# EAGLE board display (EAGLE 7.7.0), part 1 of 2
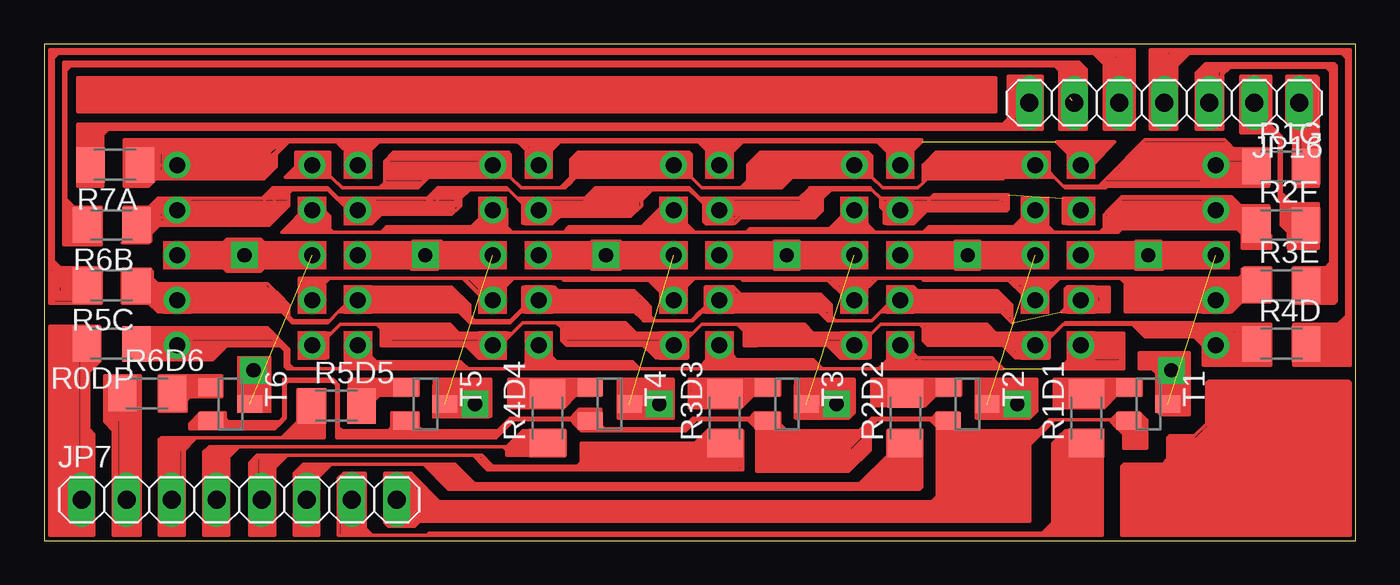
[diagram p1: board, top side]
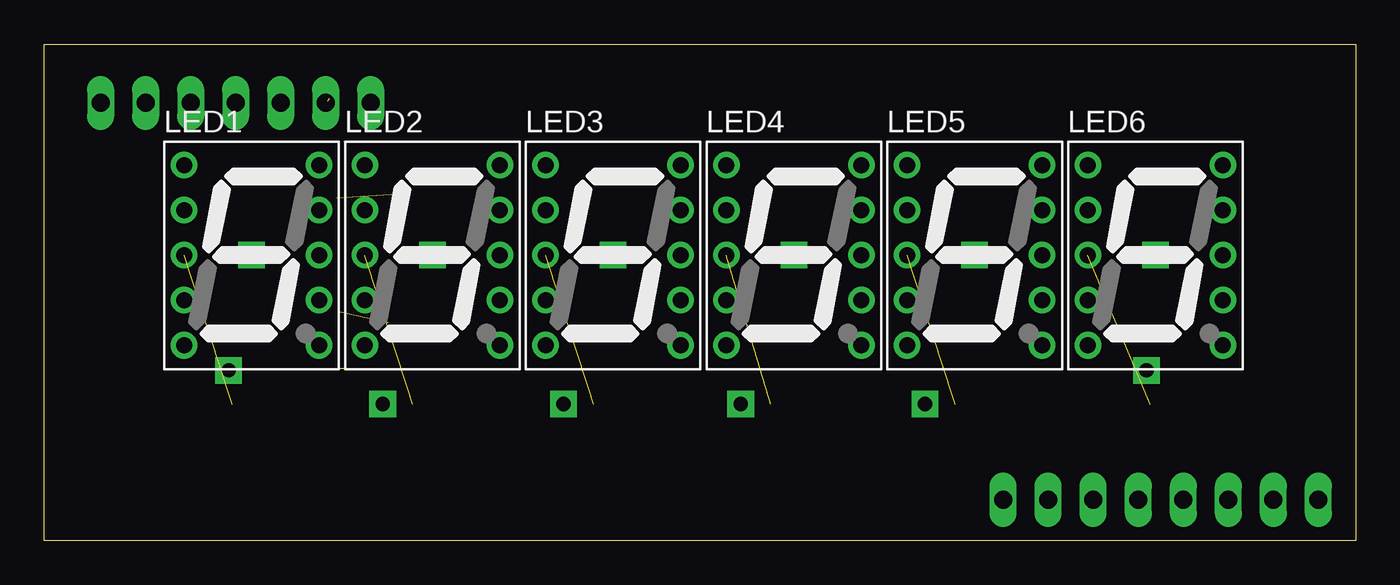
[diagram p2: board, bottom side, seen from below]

Size 74 x 28 mm. Coordinates in mm from the lower left corner, seen from the top.
Outline: 0,0 74,0 74,28 0,28 0,0
Copper layers (1*16): Top 0.035mm / dielectric 1.5mm / Bottom 0.035mm
Design rules "default": minimum track width 10mil, minimum drill 24mil, track to track 8mil, track to pad 8mil, pad to pad 8mil, via to via 8mil, smd to smd 8mil, copper to edge 40mil, drill to drill 8mil, minimum pad ring 10mil, minimum via ring 8mil, stop-mask expansion 4mil, vias tented up to drill 0mil, thermal gap 10mil

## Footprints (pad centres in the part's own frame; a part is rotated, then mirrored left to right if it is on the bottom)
1X08 = drill 1.016 long: 1 -8.89,0; 2 -6.35,0; 3 -3.81,0; 4 -1.27,0; 5 1.27,0; 6 3.81,0; 7 6.35,0; 8 8.89,0
1X07 = drill 1.016 long: 1 -7.62,0; 2 -5.08,0; 3 -2.54,0; 4 0,0; 5 2.54,0; 6 5.08,0; 7 7.62,0
SA39-11SRWA = drill 0.9 pad 1.5: 1 -3.81,5.08; 2 -3.81,2.54; 3 -3.81,0; 4 -3.81,-2.54; 5 -3.81,-5.08; 6 3.81,-5.08; 7 3.81,-2.54; 8 3.81,0; 9 3.81,2.54; 10 3.81,5.08
M1206 = smd 1.6 x 2: 1 -1.4,0; 2 1.4,0
SOT23-BEC = smd 1 x 1.4: B -0.95,-1.1; C 0,1.1; E 0.95,-1.1

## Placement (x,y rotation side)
JP7  [1X08]  11,2.3 0 top
JP16  [1X07]  63.2,24.7 180 top
LED1  SA39-11SRWA  [SA39-11SRWA]  62.3,16.1 0 bottom
LED2  SA39-11SRWA  [SA39-11SRWA]  52.1,16.1 0 bottom
LED3  SA39-11SRWA  [SA39-11SRWA]  41.9,16.1 0 bottom
LED4  SA39-11SRWA  [SA39-11SRWA]  31.7,16.1 0 bottom
LED5  SA39-11SRWA  [SA39-11SRWA]  21.5,16.1 0 bottom
LED6  SA39-11SRWA  [SA39-11SRWA]  11.3,16.1 0 bottom
R0DP  [M1206]  3.8,11.1 180 top
R1D1  4k7  [M1206]  58.8,6.9 90 top
R1G  [M1206]  69.8,21.1 0 top
R2D2  4k7  [M1206]  48.6,6.9 90 top
R2F  [M1206]  69.8,17.8 0 top
R3D3  4k7  [M1206]  38.4,6.9 90 top
R3E  [M1206]  69.8,14.4 0 top
R4D  [M1206]  69.8,11.1 0 top
R4D4  4k7  [M1206]  28.4,6.9 90 top
R5C  [M1206]  3.8,14.4 180 top
R5D5  4k7  [M1206]  16.5,7.6 0 top
R6B  [M1206]  3.8,17.8 180 top
R6D6  4k7  [M1206]  5.8,8.3 0 top
R7A  [M1206]  4,21.2 180 top
T1  [SOT23-BEC]  62.3,7.7 270 top
T2  [SOT23-BEC]  52.1,7.7 270 top
T3  [SOT23-BEC]  41.9,7.7 270 top
T4  [SOT23-BEC]  31.9,7.7 270 top
T5  [SOT23-BEC]  21.5,7.7 270 top
T6  [SOT23-BEC]  10.5,7.7 270 top

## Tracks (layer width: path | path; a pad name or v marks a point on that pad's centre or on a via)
N$1
  Top 0.2: T1.B 59.05,8.65 58.8,8.4 R1D1.2
N$2
  Top 0.2: T2.B 48.85,8.65 48.6,8.4 R2D2.2
N$3
  Top 0.2: T3.B 38.65,8.65 38.4,8.4 R3D3.2
N$4
  Top 0.2: T4.B 28.65,8.65 28.4,8.4 R4D4.2
N$5
  Top 0.2: T5.B 18.25,8.65 18,8.4 R5D5.2
N$6
  Top 0.2: 5.6,22.1 6.4,22.1 6.7,21.8 6.7,20.5 6.1,20.5 6,20.4 6,21.8 6.1,21.9 6.3,21.9 | 6.3,21.9 6.4,21.9 6.5,21.8 6.5,20.8 6.6,20.7 6.3,20.7 6.2,20.6 6.2,20.9 | 6.2,20.9 6.2,21.1 | 6.2,21.8 6.2,21.1 | 6.2,21.1 6.4,20.9 6.4,21.8 6.3,21.9 | 6.6,20.8 6.3,20.8 6.2,20.9
N$7
  Top 0.2: 30.4,8.9 26.4,8.9 26.3,9 26.3,8.8 30.2,8.8 30.3,8.7 30.3,8.6 30.2,8.5 26.5,8.5 26.4,8.6 27.8,8.6 27.9,8.7 26.3,8.7 26.2,8.6 | 26.2,8.6 26.2,9.1 31.4,9.1 31.3,9 31.4,8.9 31.4,8.2 30,8.2 29.3,7.5 26.3,7.5 26.2,7.6 26.2,7.7 | 26.2,8.6 26.2,7.7 | 26.2,7.7 26.3,7.6 27.3,7.6 27.4,7.7 26.4,7.7 26.3,7.8 27.4,7.8 27.4,7.9 27.5,8 26.3,8 26.3,8.2 27.5,8.2 27.5,8.3 26.3,8.3 26.3,8.4 26.4,8.5 30,8.5 30.1,8.4 29.4,8.4 29.3,8.3 29.3,8.2 | 29.3,7.9 29.2,7.8 29.5,7.8 30,8.3 29.8,8.3 | 29.5,8.3 29.4,8.3 29.3,8.2 | 29.3,8.2 29.3,8.1 | 29.3,8.1 29.3,7.9 | 29.3,7.9 29.4,7.9 29.8,8.3 | 29.8,8.3 29.7,8.3 | 29.7,8.3 29.5,8.3 | 29.5,8.3 29.3,8.1 | 29.3,8.1 29.5,8.1 29.7,8.3
N$9
  Top 0.2: 5.9,18.7 6,18.7 6.5,19.2 6.6,19.2 6.7,19.1 | 6.7,19.1 6.6,19.1 5.9,18.4 6,18.4 6.7,19.1 | 6.7,19.1 6.7,18.2 6.6,18.2 6,17.6 6,17.8 | 6,18 6,18.2 6.6,18.8 6.6,18.5 6.5,18.4 6.5,18.3 6,17.8 | 6,17.8 6,18 | 6,18 6.5,18.5
N$10
  Top 0.2: 12.3,22.3 13.3,22.3 13.3,22.2 | 13.3,22.2 12.6,21.5 12.6,22.2 13,22.2 | 13.3,22.2 13,22.2 | 13,22.2 12.7,21.9 | 12.7,21.9 12.7,22.1 | 12.7,21.9 12.7,21.4 | 12.7,21.4 12.6,21.3 12.6,20.8 12.5,20.7 12.5,21.5 12.7,21.5 12.9,21.7 12.9,21.1 12.7,20.9 12.7,21.4 | 12.7,21.4 12.8,21.5
N$11
  Top 0.2: R4D.1 68.4,11.02 LED1.5 66.11,11.95 65.86,12.2 61.8,12.2 | 39.5,11.27 39.75,11.02 LED3.5 46.4,11.7 46.6,11.6 | 36.1,11.27 36.15,11.02 LED4.5 29.45,11.02 29.2,11.27 29.2,12 28.9,12.3 | LED5.5 19.25,11.02 19,11.27 | 19,11.27 19,11.95 18.75,12.2 | LED6.5 15.52,11.02 15.8,11.3 | 18.75,12.2 16.7,12.2 16.2,11.7 | 16.2,11.7 16,11.5 | 16,11.5 15.8,11.3 | 15.8,11.3 15.8,11.7 16.2,11.7 | 16,11.5 16,10.3 15.8,10.3 15.7,10.4 | 18.75,12.2 22.9,12.2 23.4,11.7 26,11.7 | 19,11.27 19,11 23.8,11 24.5,10.3 26,10.3 26,11.3 27,12.3 28.9,12.3 | 25.6,11.5 25.8,11.5 26,11.7 | 26,11.7 26.2,11.7 | 26.3,11.7 26.2,11.7 | 26.2,11.7 26.1,11.6 | 28.9,12.3 32.8,12.3 33.4,11.7 | 33.5,11.6 33.4,11.7 | 33.4,11.7 36.6,11.7 | 39.5,11.3 39.5,11.27 | 35.9,11.6 36.3,11.6 | 36.3,11.6 36.4,11.6 | 39.5,11.3 39.6,11.1 45.2,11.1 45.3,11.2 39.7,11.2 39.6,11.3 44.1,11.3 45.1,10.3 45.1,10.5 44.7,10.9 45,10.9 45,10.3 44.9,10.3 44.2,11 | 39.5,11.3 39.5,11.8 | 39.5,11.8 39.5,11.9 39.1,12.2 | 29.2,12.2 32.7,12.2 33.4,11.5 34.8,11.5 34.8,11.2 33.6,11.2 | 33.6,11.2 29.5,11.2 29.4,11.3 29.4,11.5 | 29.4,11.6 29.4,11.9 29.3,12 32.6,12 32.7,12.1 32.7,12 32.8,11.9 | 32.8,11.9 33,11.7 | 29.4,11.5 33.2,11.5 33,11.7 | 29.4,11.5 29.4,11.6 | 29.4,11.6 29.5,11.7 33,11.7 | 32.8,11.9 29.5,11.9 29.5,11.4 34.8,11.4 34.9,11.3 | 33.6,11.2 34.5,10.3 36.3,10.3 36.3,10.8 | 36.3,10.8 36.1,11.1 36,11.4 36.1,11.5 36.4,11.6 | 36.4,11.6 36.2,11.4 | 36.2,11.4 36.2,11.2 | 36.2,11.2 36.3,11.1 36.3,11.3 36.2,11.5 36.2,11.4 | 36.2,11.2 36.1,11.2 | 36.1,11.2 35.5,11.2 34.7,10.4 34.6,10.4 34.1,10.9 34.7,10.9 34.8,10.8 34.8,10.7 | 34.8,10.7 34.7,10.6 34.5,10.6 34.3,10.8 34.7,10.8 34.8,10.7
  Top 0.2: 36.4,11.6 36.5,11.6 | 36.6,11.7 37.1,12.2 39.1,12.2 | 36.6,11.7 36.1,11.2 | 36.3,11.6 36.3,10.8 | 39.1,12.2 42.9,12.2 43.4,11.7 46.7,11.7 | 39.1,12.2 39.5,11.8 | 39.5,11.27 39.5,11 40.2,11 | 46.6,11.6 46.7,11.7 | 49.4,12.2 47.2,12.2 46.7,11.7 | 49.4,12.2 49.6,12 49.6,11.27 49.85,11.02 LED2.5 55.93,11 56.3,11 57,11.7 | 46.6,11.6 46.4,11.2 46.4,11.4 46.6,11.6 | 46.6,11.6 46.6,10.3 46.2,10.3 46.1,10.4 | 49.4,12.2 53.2,12.2 53.7,11.7 | 53.8,11.6 53.7,11.7 | 53.7,11.7 56.6,11.7 | 56.6,11.7 56.6,11.5 | 56.6,11.5 56.6,11.4 55.5,10.3 54.8,10.3 54.1,11 55,11 55.2,10.8 55.2,10.5 55.1,10.4 54.9,10.4 54.4,10.9 55,10.9 55.1,10.8 55.1,10.7 55,10.6 54.8,10.8 54.7,10.8 54.7,10.7 55.1,11.1 | 57,11.7 57.5,12.2 | 57.5,12.2 61.4,12.2 | 61.4,12.2 61.8,12.2 | 56.6,11.7 56.8,11.7 | 57,11.7 56.8,11.7 | 56.8,11.7 56.7,11.6 | 56.6,11.5 56.7,11.6 | 56.7,11.6 56.7,10.3 56.1,10.3 56,10.4 | 61.8,12.2 62,12 | 62.1,11.9 62.3,11.7 64.7,11.7 65.4,11 65.4,9.9 69.2,9.9 69.2,10.1 | 69.2,12.1 66,12.1 65.9,12.2 69.1,12.2 | 69.1,12.2 69.2,12.1 | 69.2,12.1 69.2,10.1 | 69.2,10.1 69.1,10 65.7,10 65.6,10.1 | 65.6,10.1 65.5,10.1 | 65.6,10.1 67.4,10.1 67.6,10.3 | 67.6,10.3 67.6,10.1 | 67.6,10.3 67.6,11.9 62.1,11.9 | 62.1,11.9 62,12 | 62,12 67.1,12 67.3,11.8 | 67.3,11.8 67.4,11.7 67.5,11.7 67.5,10.3 67.4,10.2 67,10.2 66.9,10.3 66.9,10.5 | 66.9,11.8 66.9,10.5 | 66.9,10.5 67.1,10.3 67.1,11.7 67,11.8 67,10.6 67.2,10.4 67.2,11.7 67.3,11.8 | 67.3,11.8 67.3,11.7 67.4,11.6 67.4,10.4 67.3,10.3 66.3,10.3 64.8,11.8 65,11.8 | 65.2,11.8 65.3,11.8 | 65.3,11.8 65.4,11.7 65.4,11.6 | 65.4,11.6 65.3,11.5 65,11.8 | 65,11.8 65.2,11.8 | 65.2,11.8 65.4,11.6 | 57.5,12.2 57.6,12.3 64.8,12.3 65.3,11.8
  Top 0.2: 69.1,12.2 69.2,12.2 69.2,12.1 | 61.4,12.2 62.1,11.5 65.7,11.5 65.8,11.4
N$12
  Top 0.2: 28.4,10.6 29,10
N$13
  Top 0.2: 37.8,19 37.4,19 37.2,19.2
N$14
  Top 0.2: 72.8,15.6 72.8,26.7 72.7,26.8 72.5,26.8 | 72.4,26.8 72.5,26.8 | 72.5,26.8 72.7,26.6
N$15
  Top 0.2: 38.7,10.7 38.7,10.6 39.2,10.1
N$16  (1 unrouted)
  Top 0.2: LED1.8 LED1.3
N$17  (1 unrouted)
  Top 0.2: 55.99,16.44 LED2.3 LED2.8
N$18
  Top 0.2: 13.7,12.7 13.7,13.3 13.6,13.3 | 13.6,13.3 13.6,13 | 13.6,12.8 13.6,13 | 13.6,13 6.5,13 6.1,13.4 6.3,13.4 | 6.3,13.4 13.5,13.4 13.6,13.3 | 13.6,13.3 6.4,13.3 6.3,13.4 | 6.3,13.4 6.3,13.3 6.4,13.2 13.4,13.2 13.5,13.1 13.5,13.3 12.8,14 | 12.7,14.1 12.5,14.3 6.4,14.3 6,14.7 6,14 | 6,14 6,13.8 6.1,13.7 13,13.7 | 13,13.7 13.2,13.5 | 13,13.7 12.8,13.9 6,13.9 5.9,14 6,14 | 6,14 6.1,14 | 6.1,14 12.8,14 | 12.8,14 12.7,14.1 | 12.7,14.1 6.3,14.1 6.2,14.2 6.2,14.3 6.1,14.4 6.1,14 | 6.1,14 6.3,14.2
N$19
  Top 0.2: 10.45,5.3 10.2,5.05 10.2,2.87 JP7.4 | 10.45,5.3 11,5.3 | 11,5.3 25.9,5.3 | 25.9,5.3 26.1,5.3 | 26.2,5.3 26.4,5.3 | 26.4,5.3 26.5,5.3 | 26.5,5.3 26.8,5.3 | 26.8,5.3 27.3,5.3 27.5,5.5 R4D4.1 | 9.4,5.3 9.3,5.3 9,5 9,0.8 | 9,0.8 10.4,0.8 | 10.4,0.8 10.4,4.7 11,5.3 | 10.45,5.3 9.4,5.3 | 9.4,5.3 9.1,5 9.2,5 | 9.2,5 9.3,5 | 9.3,5 9.5,5 | 9.7,5 10.5,5 | 10.5,5 10.7,5.2 9.4,5.2 9.2,5 | 10.5,5 10.3,4.8 10.3,1 10.2,0.9 10.1,0.9 10.1,4.9 9.9,4.9 9.9,0.9 9.7,0.9 9.7,5 | 9.7,5 9.5,5 | 9.5,5 9.5,0.9 9.4,0.9 9.4,4.9 9.3,5 | 9.3,5 9.3,1 9.2,0.9 9.2,5 | 9,0.8 9,0.3 10.4,0.3 10.4,0.5 | 10.4,0.8 10.4,0.5 | 10.4,0.5 10.3,0.4 9.2,0.4 9.1,0.5 9.1,0.6 10.3,0.6 | 26.1,5.3 27,6.2 29.4,6.2 29.4,4.8 26.1,4.8 26.1,5.1 25.9,5.3 | 26.1,5.3 26.2,5.3 | 26.2,5.3 27,6.1 27.3,6.1 27.3,4.9 26.4,4.9 26.2,5.1 | 26.2,5.1 26.2,5.2 | 26.2,5.1 26.2,4.9 27,4.9 27.2,5.1 27.2,5.9 27,5.9 26.4,5.3 | 26.4,5.3 26.4,5 27,5 27.1,5.1 27.1,5.8 27,5.8 26.5,5.3 | 26.5,5.3 26.5,5.1 26.9,5.1 26.9,5.5 27,5.6 27,5.5 26.8,5.3 | 26.8,5.3 26.8,5.4
N$20
  Top 0.2: 13.7,6 15.7,6 15.7,6.1 15.8,6.2 | 15.2,7.9 15.2,8.5 14.3,8.5 14.3,6.7 13.4,5.8 | 13.4,5.8 8.25,5.8 8,5.55 8,5.3 7.85,5.3 7.49,4.94 JP7.3 | 13.4,5.8 15.1,5.8 | 15.1,5.8 R5D5.1 | 15.1,5.8 15.8,5.8 15.8,6.2 | 15.8,6.2 15.8,8.5 | 15.8,6.2 14,6.2 | 14,6.2 13.7,5.9 | 14,6.2 14.4,6.6 15.7,6.6 15.7,6.3 14.2,6.3 14.4,6.5 15.5,6.5 15.6,6.4
N$21
  Top 0.2: R6D6.1 4.4,3.55 4.65,3.3 4.7,3.3 4.95,3.05 JP7.2
N$22
  Top 0.2: 14.5,21.1 14.4,21.1 13.9,20.6 14.4,20.6 14.2,20.8
N$23
  Top 0.2: 17,22.1 18.3,22.1 18.6,22.4 17,22.4 17,22.3 17.1,22.2 18.2,22.2 18.3,22.3
N$24
  Top 0.2: 5.9,17.5 6,17.5 6.5,18 6.7,18
N$25  (1 unrouted)
  Top 0.2: LED6.8 7.73,16.46 7.73,16.35 7.98,16.1 LED6.3
N$26
  Top 0.2: T6.B 8.05,8.65 7.8,8.4 R6D6.2
N$27  (1 unrouted)
  Top 0.2: 45.83,16.46 LED3.3 LED3.8
N$28
  Top 0.2: 14.8,1.3 14.8,0.8 | 14.8,0.8 14.7,0.8 | 14.7,0.8 14.1,0.8 | 14.1,0.8 14.1,3.8 14.6,4.3 15.1,4.3 | JP7.6 15.1,2.71 | 15.1,3.8 15.1,3.9 | 15.1,3.9 15.1,4.1 | 15.1,4.1 15.1,4.3 | 15.1,4.3 15.3,4.3 | 15.3,4.3 16,4.3 | 16.2,4.3 21.4,4.3 | 21.4,4.3 23.1,4.3 | 23.1,4.3 23.15,4.3 23.4,3.85 23.4,3.2 | 23.4,3.2 23.4,2.9 | 23.4,2.9 24.5,2.9 | 24.5,2.9 48.35,2.9 48.6,3.15 R2D2.1 | 15.3,4.3 15.1,4.1 | 15.1,2.71 15.1,1.2 | 15.1,1.2 14.7,0.8 | 14.8,0.8 15.5,0.8 | 15.5,0.8 15.5,3.6 16.2,4.3 | 16.2,4.3 16,4.3 | 16,4.3 15.8,4.1 14.6,4.1 14.6,4 14.3,3.7 14.3,3.8 14.4,3.9 14.4,4 14.5,4.1 15.6,4.1 15.7,4 14.8,4 14.7,3.9 14.7,3.7 | 14.7,3.7 14.7,1 14.6,0.9 14.3,0.9 14.3,3.6 14.6,3.9 15.1,3.9 | 15.1,3.9 15.5,3.9 | 15.6,3.9 15.5,3.9 | 15.5,3.9 15.4,3.8 15.4,1 15.3,0.9 15.3,1 | 15.3,1 15.3,3.5 15.6,3.8 15.2,3.8 | 15.2,3.8 15.1,3.8 | 15.1,3.8 15.1,2.71 | 15.1,1.2 15.3,1 | 15.3,1 15.1,1 15,0.9 15,3.8 15.1,3.9 | 15.1,3.9 15.2,3.8 | 15.2,3.8 15.2,1.3 15.1,1.2 | 15.1,1.2 14.9,1.2 14.9,3.8 14.8,3.8 14.7,3.7 | 14.7,3.7 14.5,3.7 14.5,1 | 14.2,1.2 14.2,0.9 14.1,0.8 | 14.1,0.8 14.1,0.3 15.5,0.3 15.5,0.5 | 15.5,0.8 15.5,0.5 | 15.5,0.5 14.2,0.5 14.2,0.6 15.3,0.6 15.4,0.7 | 21.4,4.3 22.8,2.9 23.4,2.9 | 23.1,4.3 24.5,2.9 | 24.5,2.9 24.5,3 23.2,4.3 21.8,4.3 21.7,4.2 22.9,3 24.2,3 | 24.2,3 24.2,3.1 24.1,3.2 | 24.1,3.2 23.4,3.2 | 23.4,3.2 23,3.2 22.9,3.1 22.9,3.2 21.9,4.2 23,4.2 23.9,3.3 23.7,3.3 | 23.2,3.3 23,3.3 22.2,4.1 22.9,4.1 23.7,3.3 | 23.7,3.3 23.5,3.3 | 23.3,3.3 23.2,3.3 | 23.2,3.3 22.5,4 22.8,4 23.5,3.3 | 23.5,3.3 23.3,3.3 | 23.3,3.3 22.7,3.9 | 24.2,3 46,3 47.7,4.7 | 24.1,3.2 46,3.2 47.7,4.9
N$29
  Top 0.2: 67.1,26.8 67,26.8 66.3,26.1
N$31
  Top 0.2: R2F.2 69.9,17.8 | 69.8,18 69.8,19.6 | 69.8,19.6 69.8,22.75 | 69.8,22.75 69.45,23.1 69.3,23.1 | 68.3,24.68 68.3,23.1 69.3,23.1 | 68.3,24.68 JP16.2 | 69.8,17.8 69.9,17.8 | 69.9,17.8 70.2,17.5 70.2,17.4 | 70.2,17.4 70.2,17.1 | 70.2,17.1 70.2,17 | 70.2,17 70.4,16.8 70.5,16.8 | 71.8,16.8 71.9,16.8 | 71.9,16.8 71.9,16.9 | 71.9,16.9 71.9,19 70.4,19 70.3,19.1 | 70.2,19.2 69.9,19.5 69.9,18.1 70,18 | 70,18 70.4,17.6 70.4,17.1 70.3,17 70.3,17.2 | 70.3,17.2 70.3,17.5 69.8,18 | 69.8,18 69.8,17.8 | 69.8,17.8 70.2,17.4 | 70,19.2 70,18.7 | 70,18.7 70,18 | 70,18 70.2,18 | 70.2,18 70.3,17.9 70.3,18.9 | 70.3,18.9 70.3,19.1 | 70.3,19.1 70.2,19.2 | 70.2,19.2 70.2,18.8 | 70.2,18 70.2,18.8 | 70.2,18.8 70.3,18.9 | 70.3,18.9 71.7,18.9 71.8,18.8 | 70.1,19.2 70.1,19.3 69.8,19.6 | 69.3,23.1 69.4,23 | 69.4,23 69.7,22.7 69.7,19.2 70,18.7 | 69.4,23 67.6,23 | 67.6,23 67.6,23.2 | 67.6,25.9 67.6,26.2 69.2,26.2 69.2,23.4 69.8,22.8 69.8,22.75 | 67.6,23 67.5,23 67.5,26.2 69,26.2 69.1,26.1 69.1,23.3 69.2,23.2 67.6,23.2 | 67.6,23.2 67.6,25.9 | 67.6,25.9 67.8,26.1 69,26.1 69,23.3 68,23.3 67.8,23.5 67.7,23.4 68.8,23.4 68.9,23.5 68.9,26 67.9,26 67.8,25.9 67.8,23.6 67.7,23.5 68.7,23.5 68.7,25.9 68,25.9 | 68,25.9 67.9,25.9 67.9,23.7 68.6,23.7 68.6,25.8 68.1,25.8 68,25.9 | 68,25.9 68,23.9 68.1,23.9 | 68.4,23.9 68.5,23.8 68.5,25.6 68.4,25.7 68.3,25.7 | 68.3,25.7 68.1,25.7 68.1,23.9 | 68.1,23.9 68.4,23.9 | 68.4,23.9 68.4,25.6 68.3,25.7 | 68.3,25.7 68.3,24.68 | 70.3,17.2 70.2,17.1 | 70.2,17 70.2,16.5 71.9,16.5 71.9,16.7 | 71.9,16.7 71.8,16.8 | 71.8,16.8 70.5,16.8 | 70.5,16.8 70.3,16.6 71.8,16.6 71.8,16.8 | 71.8,16.8 71.9,16.9 | 71.9,16.8 71.9,16.7
N$32
  Top 0.2: R1G.2 71.2,23.55 70.95,23.8 70.95,24.57 JP16.1
N$33
  Top 0.2: 4,1.7 4.6,1.7 4.6,1 | 4.6,0.8 3.9,0.8 | 3.9,0.8 3.9,6.2 | 3.9,6.5 3.9,6.6 | 3.9,6.6 3.9,6.8 | 3.9,6.8 3.9,7.1 3.4,7.1 | 3.4,7.1 3.4,7.4 | 3.4,7.4 3.4,9.3 3.6,9.3 | 5.2,9.3 5.2,9.2 5.4,9.2 | 5.4,9 5.4,0.8 | 5.4,0.8 4.6,0.8 | 4.6,0.8 4.6,1 | 4.6,1 4.8,1 | 4.9,1 5,1 | 5.1,1 5.2,1 | 5.2,1 5.3,1 5.3,9 5.4,9 | 5.4,9 5.4,9.2 | 5.4,9.2 5.4,9.3 5.2,9.3 | 5.2,9.3 3.6,9.3 | 3.6,9.3 3.6,7.3 | 4.1,7.3 5.2,7.3 5.2,7.1 | 5.2,7.1 3.6,7.1 3.6,7.3 | 3.6,7.3 3.7,7.3 | 3.7,7.3 4.1,7.3 | 4.1,7 4.1,0.9 4.3,0.9 4.3,6.9 4.2,6.9 4.2,7 4.1,7 | 4.1,7 4.1,7.3 | 3.6,7.3 3.5,7.3 | 3.5,7.2 3.5,7.3 | 3.5,7.3 3.4,7.4 | 3.4,7.1 3.4,6.8 | 3.4,6.8 3.4,6.7 3.9,6.2 | 3.9,6.2 3.9,6.5 | 3.9,6.5 3.6,6.8 3.6,6.9 3.5,7 3.7,7 3.9,6.8 | 3.9,6.8 4.7,6.8 | 4.7,6.8 4.9,6.8 | 4.9,6.8 5.1,6.8 5.2,6.9 5.1,7 4.6,7 4.5,6.9 4.5,1.1 4.4,1 4.6,1 | 5.2,1 5.2,7.1 | 5.2,7.1 5.1,7.2 5.1,1 | 5.1,1 5,1 | 5,1 5,6.7 4.9,6.8 | 4.9,6.8 4.9,1 | 4.9,1 4.8,1 | 4.8,1 4.7,1.1 4.7,6.8 | 3.7,7.3 3.7,6.8 3.9,6.6 | 3.9,6.6 3.6,6.6 3.4,6.8 | 3.4,6.8 3.5,6.8 4,6.3 | 3.9,0.8 3.9,0.6 | 3.9,0.6 3.9,0.4 | 3.9,0.4 5.4,0.4 | 5.4,0.4 5.4,0.5 5.4,0.6 | 5.4,0.6 5.4,0.8 | 5.4,0.6 3.9,0.6 | 3.9,0.4 3.9,0.3 5.4,0.3 5.4,0.4
N$34
  Top 0.2: R0DP.2 JP7.1
N$35  (1 unrouted)
  Top 0.2: LED4.8 LED4.3
N$36
  Top 0.2: 7,8.9 6.5,8.9 6.5,9.3 10,9.3 10,8.1 8.2,8.1 8,7.9 8,7.3 6.5,7.3 6.5,8.8 6.7,9
N$37
  Top 0.2: 7.7,9.1 9.9,9.1 9.8,9 7.8,9 | 7.7,9 7.8,9 | 7.8,9 8,8.8 8.8,8.8 8.8,8.6 8.2,8.6 8,8.4 8,8.3 | 8,8.3 7.7,8 7.9,8 8.4,8.5 8.9,8.5 8.7,8.3 8,8.3 | 7.8,8.3 8,8.3 | 8,8.3 8.2,8.5
N$38
  Top 0.2: 12.7,14.2 13.3,13.6
N$39
  Top 0.2: 45.2,11.5 39.5,11.5 39.5,11.9 39.4,12 43,12 43,11.9 43.3,11.6 39.7,11.6 39.6,11.7 43.1,11.7 42.9,11.9 39.7,11.9 39.6,11.8 39.6,11.4 39.5,11.3
N$40
  Top 0.2: 6.8,2.6 6.5,2.6 | 6.5,2.6 6.5,5.7 6.6,5.8 8.2,5.8 | 6.5,2.6 6.5,0.8 | 6.5,0.8 7.9,0.8 | 7.9,0.8 7.9,5.1 8.5,5.7 6.6,5.7 6.6,0.9 7.8,0.9 7.8,5.1 8.3,5.6 6.8,5.6 6.7,5.5 6.7,1 7,1 | 7.2,1 7.5,1 7.6,1.1 7.6,5.2 7.9,5.5 6.9,5.5 6.9,1.2 6.8,1.1 7.3,1.1 | 7.3,1.1 7.5,1.1 7.5,5.3 7.6,5.4 7.3,5.4 | 7.3,5.4 7.1,5.4 7.1,1.1 7,1 | 7,1 7.2,1 | 7.2,1 7.3,1.1 | 7.3,1.1 7.3,5.4 | 6.5,0.8 6.5,0.3 7.9,0.3 7.9,0.7 | 7.9,0.8 7.9,0.7 | 7.9,0.7 7.8,0.6 6.6,0.6 6.6,0.5 7.6,0.5 7.7,0.4 7.8,0.5
N$41
  Top 0.2: 24.5,4.7 24.9,4.3 25,4.3
N$42
  Top 0.2: 24.7,4.4 24.7,4.3 25,4 38.8,4 39.4,4.6 | 39.4,4.6 39.4,4.7 | 39.4,4.7 39.4,6.2 37.4,6.2 36.7,5.5 | 13.05,4.8 12.8,4.55 12.8,3.9 | 13.05,4.8 13.2,4.8 | 13.2,4.8 13.5,4.8 | 13.7,4.8 24.2,4.8 | 24.2,4.8 24.7,4.8 | 24.7,4.8 24.8,4.6 25.2,4.3 | 25.2,4.3 25.3,4.2 | 25.3,4.2 30.3,4.2 | 30.3,4.2 30.6,4.2 | 30.6,4.2 30.8,4.2 30.8,5.3 31,5.5 36.7,5.5 | 36.9,5.5 R3D3.1 | JP7.5 12.8,2.93 12.8,3.9 | 12.2,4.8 12,4.8 11.6,4.4 11.6,0.8 | 11.6,0.8 11.9,0.8 | 13,0.8 13,4.3 | 13,4.4 13,4.6 13.2,4.8 | 13.05,4.8 12.2,4.8 | 12.2,4.8 12,4.6 | 12,4.6 11.7,4.3 11.7,0.9 12,0.9 | 12.3,0.9 12.9,0.9 12.9,4.6 12.8,4.7 12.6,4.7 | 12.4,4.7 12.2,4.7 12.2,0.9 | 12.2,0.9 12,0.9 | 12,0.9 12,4.6 | 12,4.6 11.9,4.6 11.8,4.5 11.8,1 12.1,1 12.2,0.9 | 12.2,0.9 12.3,0.9 | 12.3,0.9 12.4,1 12.4,4.7 | 12.4,4.7 12.6,4.7 | 12.6,4.7 12.6,1.1 12.5,1 12.7,1 12.7,4.1 | 12.8,3.9 13.7,4.8 | 13.7,4.8 13.5,4.8 | 13.5,4.8 13,4.3 | 13,4.3 13,4.4 | 13,4.4 13.3,4.7 | 11.6,0.8 11.6,0.3 13,0.3 13,0.8 | 13,0.8 11.9,0.8 | 11.9,0.8 11.7,0.6 12.9,0.6 12.9,0.5 11.8,0.5 11.7,0.4 | 24.2,4.8 24.8,4.2 25.3,4.2 | 24.7,4.8 25.2,4.3 | 36.7,5.5 36.9,5.5 | 36.9,5.5 37.4,6 37.4,5.9 37.1,5.6 37.4,5.6 37.4,5.7 | 39.3,5.1 39.3,4.8 39.4,4.7 | 39.4,4.6 39.4,4 38.7,4 38.6,4.1 39.1,4.1 39.3,4.3 39.3,4.2 | 30.3,4.2 30.3,5.5 31.2,5.5 31.3,5.4 30.6,5.4 30.5,5.3 30.5,5.1 30.5,4.6 | 30.5,4.6 30.5,4.3 30.6,4.2 | 30.6,4.2 30.6,5.1 30.7,5.2 30.5,5.2 30.4,5.3 | 31,5.3 31,4.7 | 31,4.7 31,4.3 30.8,4.1 31.1,4.1 | 31,4.7 30.4,4.1 30,4.1 30.5,4.6
N$43
  Top 0.2: 15.5,14.5 15.7,14.7
N$44  (1 unrouted)
  Top 0.2: LED5.8 LED5.3
N$45
  Top 0.2: 43.9,11.4 44.9,11.4 45,11.3
N$46
  Top 0.2: 18.4,14.1 23,14.1 23.4,13.7 | 23.5,13.6 23.9,13.2 18.1,13.2 17.8,13.5 23.5,13.5 23.7,13.3 18.5,13.3 18.5,13.7 23.4,13.7 | 23.4,13.7 23.5,13.6 | 23.5,13.6 23.3,13.6 23,13.9 18.4,13.9 18.4,13.1 23.8,13.1 23.9,13 17.9,13 17.8,12.9 23.6,12.9 24.1,12.4 24.1,12.6 23.8,12.9
N$47
  Top 0.2: 2.5,4.2 2.5,1 2.6,0.9 2.3,0.9 | 1.9,0.9 2.3,0.9 | 2.3,0.9 2.4,0.8 2.8,0.8 | 2.8,0.8 2.8,4.3 | 2.8,4.3 2.8,4.4 | 2.8,4.4 2.6,4.4 | 2.6,4.4 1.9,4.4 | 1.7,4.4 1.3,4.4 | 1.3,4.4 1.3,4.2 | 1.3,4.2 1.3,0.8 | 1.3,0.8 2.6,0.8 2.7,0.9 2.7,4.3 2.3,4.3 | 2.1,4.3 1.8,4.3 | 1.8,4.3 1.5,4.3 1.5,4.2 | 1.5,4.2 1.5,0.9 2,0.9 2.1,1 2,1.1 2,4 | 2.3,0.9 2.3,4.2 | 2.3,4.2 2.3,4.3 | 2.3,4.3 2.1,4.3 | 2.1,4.3 2,4.2 2,4 | 1.8,4.3 1.8,1.1 | 2.6,3.7 2.6,4.1 2.8,4.3 | 2.8,4.4 2.8,6 2.5,6.3 2.5,9.5 3.1,10.1 3.1,12.1 1.4,12.1 | 1.4,12.1 1.4,4.3 1.5,4.2 | 1.5,4.2 1.3,4.2 | 1.3,4.4 1.3,12.1 1.5,12.1 1.6,12 1.6,4.5 1.7,4.4 | 1.7,4.4 1.9,4.4 | 1.9,4.4 1.9,10.2 2,10.3 1.8,10.3 1.8,5.1 | 1.8,5.1 1.7,5 1.7,9.9 2.1,10.3 2.1,4.1 2,4 | 2,4 2.1,4 2.3,4.2 | 2.3,4.3 2.3,6.2 2.4,6.2 2.5,6.1 2.5,4.1 2.4,4 2.4,5.6 2.7,5.9 2.7,4.8 2.6,4.7 | 2.6,4.7 2.6,4.4 | 2.6,4.7 2.6,6 2.3,6.3 2.3,10 2.4,10.1 2.3,10.1 2.2,10 2.2,9.9 2.4,9.7 2.4,9.6 3,10.2 2.6,10.2 2.5,10.1 2.5,9.8 2.7,10 2.7,10.1 | 1.8,5.1 1.8,2.7 1.9,2.6 | 1.4,1 1.4,0.9 1.3,0.8 | 1.3,0.8 1.3,0.3 | 1.3,0.3 2.8,0.3 2.8,0.6 | 2.8,0.8 2.8,0.6 | 2.8,0.6 1.4,0.6 1.4,0.5 2.7,0.5 | 1.4,12.1 0.3,12.1 0.3,0.3 1.3,0.3
N$48
  Top 0.2: 2.1,3 2.1,1.2 2.2,1.1
N$49
  Top 0.2: 1.6,4.2 1.6,1.1 1.7,1
N$50
  Top 0.2: 20.8,3.2 20.9,3.2 22.1,2 22.1,1.7 21,1.7 21,2.8 21.1,2.9 21.1,2.8 22,1.9 21.2,1.9 21.1,1.8 21.1,2.5 21.2,2.6 21.2,2.1 21.3,2 21.6,2 | 21.7,2 21.6,2 | 21.6,2 21.3,2.3 21.4,2.4 21.4,2.3 | 21.4,2.3 21.6,2.1 | 21.4,2.3 21.3,2.4 21.3,2.1
N$51
  Top 0.2: 50.4,2.1 50.4,2.2 50.8,2.6 50.8,2.5 50.4,2.1
N$52
  Top 0.2: 53.8,1.5 54.2,1.5 54.3,1.6 54.1,1.6 53.9,1.4 54.1,1.4 55.5,2.8 55.5,2.9 | 55.5,2.9 55.5,6.1 54.6,6.1 54.5,6 54.5,2.1 | 54.5,1.9 54.5,2.1 | 54.5,2.1 55.4,3 55.4,3.2 | 55.4,5.9 55.4,6 | 55.4,6 54.7,6 54.7,2.4 54.6,2.3 54.6,2.4 55.4,3.2 | 55.4,3.2 55.4,5.9 | 55.4,5.9 54.9,5.9 54.8,5.8 54.8,2.9 | 54.8,2.7 54.8,2.9 | 54.8,2.9 55.3,3.4 55.3,5.4 | 55.3,5.4 55.3,5.8 55,5.8 54.9,5.7 54.9,3.3 55,3.2 55,5.6 55.1,5.7 55.1,3.4 | 36.4,6.6 36.4,6.7 36.6,6.9 39.8,6.9 40.1,7.2 41.5,7.2 41.5,6.6 41.9,6.2 | 31.3,7.2 30.1,7.2 30.1,7.1 30,7 | 30.7,6.8 30,6.8 | 30,6.8 30,7 | 30,7 30,7.2 | 30,7.2 30.2,7.4 31.4,7.4 31.4,6.5 31.7,6.2 | 19.8,3.5 19.8,3.8 19.2,3.8 19.2,1 19.4,0.8 20.6,0.8 | 20.6,0.8 20.6,3.8 | 20.6,3.8 19.5,3.8 19.4,3.7 19.4,1 19.5,0.9 19.7,0.9 | 19.9,0.9 20,0.9 | 20.2,0.9 20.3,0.9 20.4,1 | 20.4,1 20.4,3.6 20.5,3.7 20.2,3.7 | 20.2,3.7 19.7,3.7 | 19.7,3.7 19.6,3.7 19.5,3.6 19.5,1.1 19.6,1 20.4,1 | 20.4,1 20.5,0.9 20.5,3.4 20.2,3.7 | 20.2,3.7 20.2,0.9 | 20.2,0.9 20,0.9 | 20,0.9 20,3.6 19.9,3.6 19.8,3.5 | 19.8,3.5 19.8,1 19.9,0.9 | 19.9,0.9 19.7,0.9 | 19.7,0.9 19.7,3.7 | 20.6,3.8 20.7,3.8 20.9,3.6 | 20.9,3.4 20.9,1.1 | 20.9,1.1 20.9,0.8 | 20.9,0.8 20.6,0.8 | 20.6,0.8 20.7,0.9 20.7,3.6 | 20.9,0.8 21.3,1.2 54.1,1.2 55.6,2.7 | 9.1,7 8.9,7 8.8,7.1 | 8.8,7.1 8.8,7.2 | 8.8,7.2 10.1,7.2 | 10.1,7.2 10.1,7 | 10.1,7 10.1,6.4 10.2,6.3 | 10.1,7.2 10.2,7.2 10.2,6.4 | 10.2,6.4 10.2,6.3 | 10.2,6.3 8.2,6.3 8.2,6.6 8.8,7.2 | 8.8,7.1 8.8,7 8.3,6.5 8.8,6.5 8.7,6.6 8.6,6.6 | 8.5,6.6 8.6,6.6 | 8.6,6.6 8.7,6.7 | 9.9,6.6 10.5,6.6 | 10.5,6.6 13.3,6.6 | 13.3,6.6 13.6,6.9 13.6,8.9 13.7,9 13.5,9 | 19.6,6.9 19.75,6.75 T5.E 20.4,6.45 20.57,6.28 | 20.57,6.28 20.65,6.2 | 20.65,6.2 21.2,6.2
  Top 0.2: 21.2,6.2 25.85,6.2 26.1,6.45 26.1,6.65 26.35,6.9 | 26.35,6.9 26.6,6.9 | 26.6,6.9 29.7,6.9 | 29.7,6.9 30,6.9 30.15,6.75 T4.E 30.8,6.45 31.05,6.2 31.7,6.2 | 31.7,6.2 36.05,6.2 36.3,6.45 36.3,6.55 36.55,6.8 36.8,6.8 | 41.9,6.2 41.05,6.2 40.8,6.45 T3.E 40.05,6.75 40,6.8 | 41.9,6.2 46,6.2 | 46,6.2 46.15,6.2 46.4,6.45 46.4,6.55 46.65,6.8 | 51.6,6.2 51.25,6.2 51,6.45 T2.E 50.15,6.75 50.1,6.8 50,6.8 | 51.6,6.2 52.9,6.2 | 55.6,6.2 56.3,6.2 56.5,6.4 56.5,6.6 | 36.8,6.8 39.7,6.8 | 39.7,6.8 39.9,6.8 | 46.65,6.8 46.8,6.8 | 47,6.8 50,6.8 | 56.5,6.6 56.7,6.8 57,6.8 | 60.2,6.8 60.3,6.8 60.35,6.75 T1.E | 13.5,8.75 13.5,6.95 13.25,6.7 10.2,6.7 10.15,6.75 T6.E | 13.5,8.75 13.75,9 16.25,9 16.5,8.75 16.5,6.45 | 16.5,6.45 16.75,6.2 16.8,6.2 | 16.8,6.2 19.4,6.2 | 19.4,6.2 19.5,6.2 | 19.5,6.2 19.7,6.2 | 19.7,6.2 20.4,6.2 | 20.4,6.2 20.48,6.28 20.57,6.28 | 52.65,2.2 52.9,2.45 | 52.9,2.45 52.9,6.2 | 13.5,9 13.5,8.75 | 10.2,6.3 13,6.3 13.3,6.6 | 10.2,6.4 12.9,6.4 13,6.5 | 10.5,6.6 10.1,7 | JP7.8 20.6,2.3 20.6,1.5 52.9,1.5 52.9,2.45 | 55.6,2.7 55.6,5.6 | 55.6,5.6 55.6,6.2 | 55.6,6.2 52.9,6.2 | 51.6,6.2 51.6,7.2 50.4,7.2 50.1,6.9 50.1,6.7 | 50.1,6.7 50.3,6.5 | 50.3,6.9 50.3,6.5 | 50.3,6.5 50.4,6.4 | 50.4,6.4 50.5,6.3 50.5,2.4 50.3,2.2 22.3,2.2 20.9,3.6 | 20.9,3.6 20.9,3.4 | 20.9,3.4 22.2,2.1 22.2,1.4 21,1.4 21,1.1 21.2,1.3 22.2,1.3 22.3,1.4 | 20.65,6.2 20.4,6.2 | 19.7,6.2 19.7,7.2 | 19.7,7.2 19.6,7.2 19.6,6.3 19.5,6.2 | 19.7,7.2 21.1,7.2 21.1,6.3 21.2,6.2 | 16.5,6.45 16.5,5.8 25.5,5.8 26.1,6.4 | 19.9,6.5 19.7,6.5 19.4,6.2 | 25.7,6.1 25.8,6.1 26.6,6.9 | 16.6,6.2 16.6,6.1 | 16.6,6.1 16.6,6 25.5,6 25.6,6.1 25.5,6.1 | 25.5,6.1 21.4,6.1 | 21.4,6.1 16.6,6.1 | 20.9,6.6 21.4,6.1
  Top 0.2: 26.35,6.9 26.3,6.9 25.5,6.1 | 30,6.8 30,6.7 | 30,6.5 30.3,6.2 36.2,6.2 36.8,6.8 | 39.7,6.8 40.2,6.3 | 40.2,6.3 40.5,6 40.7,6 | 40.7,6 40.9,6.2 | 40.9,6.2 40.5,6.2 | 40.5,6.2 39.9,6.8 | 39.9,6.8 40,6.8 | 40,6.8 40.2,7 | 40.7,6 46.2,6 46.6,6.4 | 47,6.8 46.9,6.8 | 46.9,6.8 46.8,6.8 | 46.8,6.8 46.6,6.6 | 46.6,6.6 46.3,6.3 46.4,6.3 46.9,6.8 | 46.65,6.8 46.6,6.8 | 46.6,6.8 46,6.2 | 40.9,6.2 41.1,6.2 41.2,6.1 | 46.6,6.6 46.6,6.8 | 46.6,6.8 46.7,6.9 50.7,6.9 | 50,6.8 50.1,6.7 | 50.4,6.4 50.4,2.5 50,2.1 | 55.4,6 55.9,6 | 55.9,6 56.2,6 | 56.2,6 56.4,6.2 | 56.4,6.2 56.9,6.7 | 56.9,6.7 57,6.8 | 56.5,6.6 55.9,6 | 55.9,6 55.3,5.4 | 55.3,5.4 55.6,5.4 56.2,6 | 56.4,6.2 56.2,6.2 55.6,5.6 | 55.5,2.9 55.4,2.9 54.6,2.1 54.6,2.5 55,2.9 | 40.4,6.8 40.4,6.5 40.2,6.3 | 40.2,6.3 40.2,3.9 45.4,3.9 46.6,5.1 46.6,6.4 | 46.6,6.4 47,6.8 | 40.5,6.2 40.3,6 | 20.8,1.2 20.9,1.1 | 20.9,1.1 55.6,1.1 55.6,1.7 | 55.6,2.4 55.6,2.6 | 55.6,2.7 55.6,2.6 | 55.6,2.6 54.2,1.2 55.4,1.2 55.5,1.3 55.5,2.2 55.3,2.2 54.4,1.3 54.5,1.3 55.6,2.4 | 55.6,2.4 55.6,1.7 | 55.6,1.7 55.3,1.4 54.8,1.4 | 54.8,1.4 54.7,1.3 | 54.8,1.4 55.4,2 55.4,1.6 55.3,1.5 55.3,1.6 55.2,1.7 55.3,1.7 55.1,1.5 55.3,1.3 | 56.9,6.7 56.8,6.7 56.6,6.5 | 57,6.8 60.2,6.8 | 60.3,6.9 60.6,7.2 61.8,7.2 62.1,6.9 | 62.1,6.9 60.3,6.9 | 60.3,6.9 60.2,6.8 | 60.2,6.8 60.2,6.7 60.5,6.4 | 60.6,6.3 60.6,6.5 60.5,6.6 60.5,6.4 | 60.5,6.4 60.6,6.3 | 60.6,6.3 60.9,6 60.9,5.2 62.2,5.2 62.2,6.8 62.1,6.9 | 62.1,6.9 62,6.8 62,5.3 61.1,5.3 61,5.4 61,6.1 60.9,6.2 61.8,6.2 61.9,6.3 61.9,5.5 61.8,5.4 61.3,5.4 61.2,5.5 | 61.2,5.5 61.2,5.7 | 61.2,5.9 61.2,6.1 61.4,6.1 | 61.4,6.1 61.6,6.1 | 61.6,6.1 61.7,6 61.7,5.8 | 61.7,5.8 61.4,5.5 | 61.4,5.5 61.3,5.5 61.2,5.4 61.2,5.5
  Top 0.2: 61.2,5.8 61.2,5.9 | 61.2,5.9 61.4,6.1 | 61.6,6.1 61.7,6.1 61.8,6 61.8,5.7 | 61.8,5.7 61.8,5.5 61.4,5.5 | 61.4,5.5 61.2,5.7 | 61.2,5.7 61.2,5.8 | 61.2,5.8 61.4,6 61.5,6 61.7,5.8 | 61.3,5.8 61.7,5.8 | 61.7,5.8 61.8,5.7 | 61.8,5.7 61.7,5.6 61.4,5.6 61.3,5.7 | 26.4,6.8 29.7,6.8 30,6.5 | 30,6.5 30,6.7 | 30,6.7 29.9,6.8 29.8,6.8 29.7,6.9 | 29.7,6.9 30,7.2 | 13.5,9 13.5,9.1 16.3,9.1 16.6,8.8 16.6,6.4 16.8,6.2
N$53
  Top 0.2: 51.1,5.9 50.7,6.3 51,6.3 51.1,6.2
N$54
  Top 0.2: 50.7,5.9 50.7,6.1 50.6,6.2
N$55
  Top 0.2: 18.1,8.2 18.3,8.2 18.4,8.3 18.4,8.2 21.1,8.2 21.1,9.1 17.2,9.1 17.2,6.7 18.6,6.7 18.6,8.1 18.8,8.3 19.6,8.3 19.7,8.4 19.7,8.5 | 19.7,8.5 19.7,8.8 | 19.7,8.8 19.6,8.9 | 19.6,8.9 17.3,8.9 | 19.6,8.9 19.8,8.9 19.9,8.8 19.7,8.8 | 19.7,8.8 19.6,8.7 17.3,8.7 17.3,8.5 18.8,8.5 | 19.7,8.5 19.6,8.5 19.4,8.5 | 19.4,8.5 18.8,8.5 | 18.8,8.5 18.6,8.3 19.2,8.3 19.4,8.5 | 19.4,8.5 19.2,8.5 18.5,7.8
N$56
  Top 0.2: 22.9,8.2 22.3,8.2 22,8.5 | 22,8.5 22,9.1 23.8,9.1 | 25,9.1 23.8,9.1 | 23.8,9.1 22,7.3 | 22,7.3 22,7 25.2,7 25.2,9.1 25,9.1 | 25,9.1 25,9 25.1,8.9 22.1,8.9 | 22,8.5 22,7.3
N$57
  Top 0.2: 39.1,4.9 39,4.9 38.6,4.5 38.8,4.5 39,4.7 39.2,4.7 38.7,4.2 38.9,4.2 39.3,4.6
N$58
  Top 0.2: 47.3,4.4 47.6,4.7 47.6,6.2 49.5,6.2 49.5,3.4 | 49.5,3.4 49.5,3.2 | 49.5,3.2 49.5,3 49.4,2.9 49.2,2.9 | 48.8,2.9 49.2,2.9 | 49.2,2.9 49.4,3.1 49.4,4.2 | 49.4,4.2 49.4,4.6 49.3,4.7 47.9,4.7 47.8,4.6 47.7,4.6 | 47.7,4.6 47.6,4.5 | 47,3.9 46.3,3.2 | 46.3,3.2 46.1,3 47.7,3 | 47.7,3 49.3,3 49.5,3.2 | 49.5,3.2 49.3,3.2 | 46.3,3.2 49.3,3.2 | 49.3,3.2 49.5,3.4 | 49.5,3.4 46.7,3.4 | 46.7,3.4 46.6,3.3 | 46.7,3.4 46.9,3.6 49.3,3.6 49.3,3.4 48.8,2.9 | 48.8,2.9 47.8,2.9 47.7,3 | 47.7,3 47,3.7 49.2,3.7 49.3,3.8 49.3,3.9 | 49.3,4.3 49.3,4.5 47.6,4.5 | 47.6,4.5 47,3.9 | 47,3.9 47.2,3.9 | 47.2,3.9 49.3,3.9 | 49.3,3.9 49.3,4.1 | 49.3,4.1 49.4,4.2 | 49.4,4.2 47.5,4.2 | 47.5,4.2 47.4,4.2 47.3,4.1 49.3,4.1 | 49.3,4.1 49.3,4.3 | 49.3,4.3 47.8,4.3 47.7,4.4 | 47.7,4.4 47.5,4.2 | 47.7,4.6 47.7,4.4 | 47.5,4.2 47.2,3.9
N$59
  Top 0.2: 31.5,6.3 36,6.3 36.5,6.8
N$60
  Top 0.2: 33.2,8.1 32.7,8.1 32.4,8.4 32.4,9.1 32.5,9.1 | 32.5,9.1 35.5,9.1 35.5,7.3 | 35.5,7.3 35.5,7.1 | 35.5,7.1 35.4,7 32.4,7 32.4,8.8 32.5,8.9 35.4,8.9 35.4,7.7 35.2,7.5 35.3,7.5 35.5,7.3 | 35.5,7.1 35.5,6.9 32.4,6.9 32.4,9 32.5,9.1
N$61
  Top 0.2: 16,11.6 15.9,11.6
N$62
  Top 0.2: 36.5,9 40.1,9 40.2,8.9 36.5,8.9 36.4,8.8 | 38.2,8.7 37.9,8.7 37.5,9.1 | 37.5,9.1 36.4,9.1 36.4,8.8 | 36.4,8.8 36.4,7.5 39.1,7.5 | 39.9,8.3 39.1,7.5 | 39.1,7.5 39.3,7.5 40,8.2 41.5,8.2 41.5,9.1 37.5,9.1 | 37.5,9.1 37.4,9 | 36.4,8.8 40.4,8.8 40.5,8.9 40.5,8.8 40.2,8.5 36.6,8.5 36.5,8.6 37.5,8.6 37.6,8.7 39.9,8.7 40.3,8.3 39.7,8.3 | 37,8.3 36.7,8.3 36.6,8.4 36.6,7.6 39,7.6 39.7,8.3 | 39.7,8.3 37,8.3 | 37,8.3 36.7,8 37.5,8 37.7,7.8 37.7,8 37.6,8.1 36.9,8.1 36.8,8.2 36.8,7.8 37.4,7.8 37.5,7.7 36.7,7.7
N$63
  Top 0.2: 19.1,12 19,12.1 19.1,12.1 19.2,12 19.2,11.2 19.3,11.2 19.3,11.6 | 19.3,11.6 19.3,12 22.9,12 22.9,11.9 | 22.9,11.9 22.9,11.8 19.4,11.8 19.4,11.7 19.3,11.6 | 19.3,11.6 23.2,11.6 | 23.3,11.6 23.2,11.6 | 23.2,11.6 22.9,11.9 | 22.9,11.9 23,11.9 23.2,11.7 19.7,11.7 19.4,11.4 19.6,11.4 | 19.9,11.4 24.7,11.4 24.7,11.6 20.1,11.6 19.9,11.4 | 19.9,11.4 19.6,11.4 | 19.6,11.4 19.4,11.2 24.5,11.2
N$64
  Top 0.2: 41.4,6.7 41.4,6.6 41.7,6.3
N$65
  Top 0.2: 42.8,8.4 42.8,8.7 42.6,8.9 | 42.6,8.9 42.5,9 | 42.4,9.1 45.7,9.1 45.7,7.2 45.4,6.9 42.4,6.9 42.5,9 | 42.5,9 42.4,9.1 | 42.4,9.1 42.4,7.4 42.5,7.3 | 42.6,8.9 45.5,8.9
N$66
  Top 0.2: 45.5,9 45.5,7.2
N$67
  Top 0.2: 48.5,8.8 48.5,9.1 46.7,9.1 46.7,8.1 | 46.7,8.1 46.7,7.6 49.7,7.6 50.5,8.4 50.4,8.4 50.2,8.2 51.7,8.2 51.7,9.1 48.1,9.1 48,9 | 48,9 46.9,9 | 48,9 50.3,9 50.4,8.9 46.8,8.9 46.8,8.7 50.6,8.7 50.6,8.5 46.8,8.5 46.8,8.3 50.5,8.3 50.6,8.4 50.3,8.4 50,8.1 46.7,8.1 | 46.7,8.1 46.8,8 49.9,8 | 50,8 49.9,8 | 49.9,8 49.7,7.8 46.8,7.8
N$68
  Top 0.2: 53.8,8 52.7,9.1 | 52.7,9.1 52.6,9.1 52.6,6.9 55.6,6.9 56,7.3 56,9 52.7,9 52.7,9.1 | 52.7,9.1 56,9.1 56,8.5 55.9,8.4 55.9,8.9 52.9,8.9 52.8,8.8 52.7,8.9 55.7,8.9 55.8,8.8 55.8,7.3 55.6,7.1 55.6,7.6
N$69
  Top 0.2: 40.4,7 40,7 39.9,6.9
N$70
  Top 0.2: 39.9,6.7 40.4,6.2
N$71  (via drill 0.8 pad 1.5)
  other vias: 11.8,9.6
N$72  (via drill 0.8 pad 1.5)
  other vias: 24.3,7.7
N$73  (via drill 0.8 pad 1.5)
  other vias: 34.7,7.7
N$74  (via drill 0.8 pad 1.5)
  other vias: 44.7,7.7
N$75  (via drill 0.8 pad 1.5)
  other vias: 54.9,7.7
N$76  (via drill 0.8 pad 1.5)
  other vias: 63.6,9.6
N$77  (via drill 0.8 pad 1.5)
  other vias: 62.3,16.1
N$78  (via drill 0.8 pad 1.5)
  other vias: 52.1,16.1
N$79  (via drill 0.8 pad 1.5)
  other vias: 41.9,16.1
N$80  (via drill 0.8 pad 1.5)
  other vias: 31.7,16.1
N$81  (via drill 0.8 pad 1.5)
  other vias: 21.5,16.1
N$82  (via drill 0.8 pad 1.5)
  other vias: 11.3,16.1
N$83
  Top 0.2: 40.3,5.9 45.4,5.9 | 45.4,5.9 46.3,5.9 46.5,6.1 45.6,6.1 45.4,5.9 | 45.4,5.9 45.4,5.4 | 45.4,5.2 45.4,4.9 | 45.4,4.9 45.4,4.1 | 45.4,4.1 45.3,4 | 45.4,4.1 46.5,5.2 46.5,5.4 | 46.5,6 46.5,5.4 | 46.5,5.4 45.5,4.4 45.5,4.6 46.4,5.5 46.3,5.5 45.5,4.7 45.5,4.8 46.4,5.7 46.2,5.7 | 46.2,5.7 45.4,4.9 | 46.2,5.7 46.4,5.9 46.1,5.9 45.4,5.2 | 45.4,5.2 45.4,5.4 | 45.4,5.4 45.7,5.7 45.8,5.7 45.9,5.8 45.6,5.8 45.5,5.7
N$84
  Top 0.2: 59.2,8.7 59.2,9.1 | 59.2,9.1 57.4,9.1 | 57.4,9.1 57,9.1 57,7.5 59.8,7.5 60.5,8.2 61.9,8.2 61.9,9.1 59.2,9.1 | 57.4,9.1 57.2,8.9 | 57.2,8.9 57.1,8.9 | 57.2,8.9 61,8.9 61.1,8.8 57.2,8.8 57.1,8.7 60.4,8.7 60.6,8.5 57.2,8.5 57.1,8.4 57.3,8.4 | 60.8,8.4 57.3,8.4 | 57.3,8.4 57.1,8.6 57.1,8.2 60.3,8.2 | 60.3,8.2 60.4,8.3 | 60.3,8.2 59.8,7.7 59.8,7.9 60,8.1 57.2,8.1 57.1,8 57.1,7.8 | 57.1,7.8 57.1,7.6 57.3,7.6 | 57.9,7.6 57.3,7.6 | 57.3,7.6 57.1,7.8 | 57.1,7.8 57.9,7.8 57.9,8 57.3,8 57.2,7.9
N$85
  Top 0.2: 58.9,4.9 58.9,6.1 58.8,6.2 57.6,6.2 57.3,5.9 | 57.3,5.9 57.3,5.8 56.9,5.4 | 56.9,5.4 56.9,5.5 57.3,5.9 | 56.9,5.4 56.9,0.9
N$86
  Top 0.2: 59.6,6.2 59.7,6.2 59.7,0.4 | 17.6,0.4 17.6,3.6 17.7,3.7 17.4,3.7 17.4,0.4 17.2,0.4 17.2,3.8 | 17.5,3.2 17.5,3.8 | 17.5,3.8 17.4,3.8 | 17.4,3.8 17.2,3.8 | 17.1,3.8 16.9,3.8 16.6,3.5 16.6,0.3 17.5,0.3 | R1D1.1 58.8,0.55 58.55,0.3 | JP7.7 17.5,1.95 17.5,0.3 | 17.5,0.3 18,0.3 | 18,0.3 18.2,0.3 | 18.5,0.3 21.6,0.3 | 21.6,0.3 56.4,0.3 | 56.4,0.3 58.5,0.3 | 18,0.3 18,0.5 | 18,0.5 18,3.2 | 18,3.2 17.4,3.8 | 17.5,3.8 18.1,3.8 18.1,0.7 18.5,0.3 | 18.5,0.3 18.3,0.3 | 18.3,0.3 18.2,0.3 | 18.2,0.3 18,0.5 | 18,0.5 17.9,0.5 17.8,0.4 17.8,0.8 | 17.8,0.8 17.8,3.7 17.9,3.6 18,3.7 18,3.2 | 17.2,3.8 17.1,3.8 | 17.1,3.8 17,3.7 17,0.4 16.8,0.4 16.8,3.5 | 17.8,0.8 18.3,0.3 | 59.7,0.4 58.6,0.4 | 58.6,0.4 58.5,0.3 | 58.55,0.3 59.6,0.3 | 59.6,0.3 59.7,0.4 | 59.7,0.4 59.7,0.3 59.6,0.3 | 58.55,0.3 58.5,0.3 | 56.4,0.3 57.1,1 57.1,0.8 56.7,0.4 58.6,0.4 | 21.6,0.3 21.7,0.4 56.3,0.4 57,1.1
N$87
  Top 0.2: 58,6 57.5,6 57.5,5.9 57.2,5.6 57.9,5.6 57.9,5.7 | 57.9,5.7 57.9,5.8 58,5.9 57.6,5.9 57.4,5.7 | 57.9,5.7 57.4,5.7 | 57.4,5.7 57.1,5.4
N$88
  Top 0.2: 55,3 55.1,3 55.3,3.2 55,3.2 54.9,3.1
N$89
  Top 0.2: 23.9,11 24.3,10.6 | 24.3,10.6 24.5,10.4 24.5,10.6 | 24.5,10.7 24.4,10.8 24.4,10.9 24.1,10.9 24.2,10.8 24.7,10.8 24.5,10.6 | 24.3,10.6 24.5,10.6
N$90
  Top 0.2: 10.1,15.6 10.3,15.6 10.6,15.3 11.9,15.3 12.1,15.5
N$91
  Top 0.2: 8.2,10.8 10,10.8 10.1,10.9 8.1,10.9 8.1,10.7 8.4,10.7 | 9.8,10.7 8.4,10.7 | 8.4,10.7 8.2,10.5 9.7,10.5 9.8,10.6 9.7,10.6 9.4,10.3 8.2,10.3
N$92
  Top 0.2: 9.9,15.7 9.9,15.6 10.3,15.2 12.2,15.2 12.5,15.5
N$93
  Top 0.2: 15.4,21.8 15.6,21.8 | 15.6,21.8 15.7,21.9 15.8,21.9 | 15.8,21.9 15.9,21.9 | 15.5,20.8 15.8,20.8 15.9,20.7 | 15.9,21.9 15.9,20.7 | 15.9,20.7 16,20.6 | 15.6,21.8 15.7,21.8 15.8,21.9 | 15.9,21.9 16.1,21.9 16.1,20.6 16.2,20.5 | 14.6,21.9 14.2,21.9 14.2,21.1 13.6,20.5 16.2,20.5 | 16.2,20.5 16.5,20.2
N$94
  Top 0.2: 9.8,16.5 10.3,17 12.2,17 12.4,16.8
N$95
  Top 0.2: 20.2,15.6 20.4,15.6 20.7,15.3 22.2,15.3 22.5,15.6
N$96
  Top 0.2: 20.2,16.4 20.3,16.4 20.8,16.9 22.4,16.9 22.8,16.5
N$97
  Top 0.2: 30.6,16.6 30.9,16.9 32.5,16.9 32.8,16.6
N$98
  Top 0.2: 30.5,15.8 30.5,15.7 30.9,15.3 32.5,15.3 32.9,15.7
N$99
  Top 0.2: 40.6,16.4 40.7,16.4 41.2,16.9 42.6,16.9 43,16.5
N$100
  Top 0.2: 40.5,15.7 40.8,15.7 41.2,15.3 42.6,15.3 43.1,15.8
N$101
  Top 0.2: 50.8,16.3 51.4,16.9 52.8,16.9 53.4,16.3
N$102
  Top 0.2: 51.1,15.8 51.1,15.6 51.4,15.3 52.8,15.3 53.4,15.9
N$103
  Top 0.2: 61.2,16.6 61.3,16.6 61.6,16.9 63,16.9 63.4,16.5
N$104
  Top 0.2: 60.7,15.7 61.2,15.7 61.6,15.3 63.1,15.3 63.8,16
N$105
  Top 0.2: 7.7,19.3 6.4,19.3 5.9,18.8 4.5,18.8 4.5,16.9 4.4,16.8 5.9,16.8 6,16.9 6,17.3 6.5,17.8 12.7,17.8 13.6,18.7
N$106
  Top 0.2: 38.3,18.1 38.5,18.1 38.7,17.9 39,17.9 39.3,18.2 43.5,18.2 43.9,18.6 43.9,19.3 44.4,19.8 | 38.6,19.1 38.7,19.3 42.6,19.3 43.1,19.8 | 43.1,19.8 44.4,19.8 | 44.4,19.8 46.7,19.8 | 46.7,19.8 47.3,19.2 | 47.4,19.1 47.7,19.1 47.7,19.3 47.3,19.3 47.3,19.2 | 47.3,19.2 47.4,19.1 | 47.4,19.1 47.4,17.9 49,17.9 49.6,18.5 49.4,18.5 49.1,18.2 49.1,18.6 | 49.1,18.9 49.1,18.6 | 49.1,18.6 49.2,18.5 49.2,18.6 49.4,18.8 49.3,18.8 49.2,18.7 50.1,18.7 50.2,18.8 | 50.2,18.8 49.7,18.8 | 50.2,18.8 54.2,18.8 54.2,19.1 54.1,19.2 | 43.1,19.8 43.2,19.9 46.6,19.9 46.7,19.8
N$107
  Top 0.2: 34.9,14.2 34.7,14.2 34.6,14.3
N$108
  Top 0.2: 28.8,14.2 28.8,13.8 | 28.8,13.8 28.8,13.7 28.7,13.6 33.4,13.6 33.5,13.7 33.2,14 28.8,14 28.7,14.1 28.7,13.9 28.8,13.8 | 28.8,13.8 33.3,13.8 33.4,13.7
N$109
  Top 0.2: 48.7,14.2 48.8,14.3
N$110
  Top 0.2: 28.7,13.1 33.3,13.1 33.8,12.6 34,12.6 34.1,12.7 34.1,13.2 | 34.1,13.2 33.8,13.5 33.5,13.5 33.4,13.4 33.4,13.2 | 33.4,13.2 33.9,12.7 33.9,13.1 33.6,13.4 33.6,13.2 33.8,13 33.9,13 34,13.1 | 34,13.1 34.1,13.2 | 34.1,13.2 33.4,13.2 | 33.4,13.2 33.3,13.3 28.6,13.3 | 28.5,13.7 28.5,13.2 | 28.5,13.2 28.5,13 28.6,12.9 33.3,12.9 33.7,12.5 | 33.7,12.5 34.3,12.5 34.4,12.4 33.8,12.4 33.7,12.5 | 28.6,13.3 28.5,13.2 | 28.6,13.3 28.8,13.5 33.2,13.5 33.3,13.4 | 33.7,13.4 34,13.1
N$111
  Top 0.2: 48.9,13 48.9,12.9 54,12.9 54.5,12.4
N$112
  Top 0.2: 8,19.3 12.3,19.3 12.9,19.9 16,19.9 16.3,19.6
N$113
  Top 0.2: 48.9,13.3 54.5,13.3
N$114
  Top 0.2: 48.9,13.4 54.3,13.4
N$115
  Top 0.2: 48.7,13.8 54,13.8 54.1,13.7 48.9,13.7 48.9,13.8 49,13.9 49.2,13.9 | 53.9,13.9 49.4,13.9 | 49.4,13.9 49.2,13.9 | 49.2,13.9 49,14.1 | 49.1,14.2 49.4,13.9
N$116
  Top 0.2: 49.8,11.2 55.1,11.2 55.2,11.3 49.9,11.3 49.8,11.4 | 49.8,11.4 49.7,11.4 | 49.8,11.4 55.4,11.4 55.5,11.5 55.4,11.5 55.3,11.6 50,11.6 | 50,11.6 49.9,11.6 49.8,11.5 49.8,11.9 49.7,12 53.2,12 | 53.2,12 53.2,11.9 53.4,11.7 | 53.4,11.7 53.5,11.7 | 53.4,11.7 50,11.7 49.9,11.8 53.2,11.8 | 50,11.6 49.7,11.3 | 53.2,12 53.4,11.8
N$117
  Top 0.2: 54.9,11.1 54.9,10.5 55.1,10.5
N$118
  Top 0.2: 48.7,10.8 48.8,10.8 49.4,10.2
N$119  (1 unrouted)
  Top 0.2: 58.5,11.2 58.5,11.7 60.9,11.7 60.9,9.8 60.6,9.8 | 13.4,11 12.9,11.5 | 12.8,11.6 12.6,11.8 8.1,11.8 | 5.1,12 8.1,12 | 8.1,12 8.3,12 | 8.3,12 8.3,11.4 | 8.3,11.4 8.3,10.2 | 8.3,10.2 4.5,10.2 4.5,11.9 8,11.9 | 8,11.9 8.1,11.8 | 8.1,11.8 8.2,11.7 | 8.2,11.9 8.2,11.7 | 8.2,11.7 8.1,11.6 | 8.1,11.6 4.7,11.6 4.8,11.7 8.1,11.7 | 8.1,11.7 8.1,11.6 | 8.1,11.6 8.1,11.4 8,11.3 5.2,11.3 | 5.1,11.3 5.2,11.3 | 5.2,11.3 5.4,11.5 7.4,11.5 7.5,11.4 7.5,11.2 7.3,11 5.3,11 R0DP.1 | LED1.6 58.5,9.7 | 58.5,9.7 57.4,9.7 | 57.4,9.7 57.3,9.7 57.4,9.8 | 53.9,9.7 49.5,9.7 | 49.3,9.7 48.3,9.7 | 48.3,9.7 48.29,9.7 | 48.29,9.7 LED2.6 48.3,9.7 | 48.29,9.7 47.6,9.7 | 47.2,9.7 47.1,9.7 | 47.1,9.7 43.9,9.7 | 43.7,9.7 39.2,9.7 | 39.1,9.7 38.1,9.7 | 38.1,9.7 38.09,9.7 | 38.09,9.7 LED3.6 38.1,9.7 | 38.09,9.7 36.9,9.7 | 36.9,9.7 33.6,9.7 | 33.6,9.7 28.9,9.7 | 28.8,9.7 28.3,9.7 | 28.3,9.7 27.9,9.7 | 27.89,9.7 LED4.6 27.9,10.1 | 27.9,10.1 27.9,9.7 | 27.89,9.7 26.9,9.7 | 26.9,9.7 23.9,9.7 | 23.9,9.7 18.7,9.7 | 18.6,9.7 17.7,9.7 | 17.7,9.7 17.69,9.7 | 17.69,9.7 LED5.6 17.7,9.7 | R0DP.1 5.2,11.02 LED6.6 13.55,11.02 13.8,10.77 13.8,9.95 14.05,9.7 16.7,9.7 | 16.7,9.7 17.69,9.7 | R0DP.1 7.2,11.1 7.3,11.2 7.3,10.8 5.9,10.8 5.9,10.7 5.8,10.6 7.2,10.6 7.2,10.4 5.6,10.4 | 8,11.9 8.1,12 | 8.3,12 12.6,12 13.8,10.8 | 8.3,10.2 9.5,10.2 10.3,11 13.3,11 13.6,10.7 13.6,9.9 | 13.6,9.9 13.6,9.8 13.7,9.7 13.8,9.7 | 14,9.7 13.8,9.7 | 13.8,9.7 13.6,9.9 | 8.1,11.8 8.1,11.7 | 8.1,11.6 12.8,11.6 | 12.8,11.6 12.9,11.5 | 12.9,11.5 12.9,11.4 13.1,11.2 8.3,11.2 8.2,11.3 8.3,11.4 | 8.3,11.4 12.8,11.4 | 16.7,9.7 17,10 17,11.7 18.4,11.7 18.4,10 18.7,9.7 | 18.7,9.7 18.6,9.7 | 18.6,9.7 18.4,9.9 | 18.4,9.9 17.1,9.9 17,9.8 17,9.9 17.2,10.1
  Top 0.2: 17.2,10.1 17.1,10.2 | 27.2,10.4 27.2,10 26.9,9.7 | 27.89,9.7 27.9,9.7 | 28.3,9.7 27.9,10.1 | 28.3,10.1 28.4,10.1 | 28.4,10.1 28.6,10.3 28.6,10 28.9,9.7 | 28.9,9.7 28.8,9.7 | 28.8,9.7 28.5,10 27.3,10 27.2,9.9 27.9,9.9 | 28.5,9.9 27.9,9.9 | 27.9,9.9 27.6,10.2 | 27.6,10.2 27.3,10.2 | 27.6,10.2 27.8,10.2 27.9,10.1 | 27.9,10.1 28.3,10.1 | 28.3,10.1 28.5,9.9 | 28.5,9.9 28.6,9.8 | 36.9,9.7 37.5,10.3 38.7,10.3 | 38.7,10.3 38.8,10.3 | 38.8,10.3 38.8,10.1 | 38.8,10.1 39.1,9.8 | 39.1,9.8 39.2,9.7 | 39.2,9.7 39.1,9.7 | 39.1,9.7 39,9.8 | 39,9.8 38.9,9.9 37.3,9.9 37.5,10.1 | 37.5,10.1 38.7,10.1 | 37.5,10.1 37.4,10.1 37.2,9.9 37.2,9.8 | 39,9.8 38.9,9.8 38.7,10 | 38.7,10.3 38.7,10.2 38.8,10.1 | 38.8,10.5 38.8,10.3 | 47.6,10.4 47.6,9.7 | 47.6,9.7 47.2,9.7 | 47.2,9.7 47.7,10.2 47.7,10 47.5,9.8 | 47.1,9.7 47.8,10.4 | 49,10.4 49,10.3 | 49,10.3 49,10.2 49.3,9.9 | 49.3,9.9 49.5,9.7 | 49.5,9.7 49.3,9.7 | 49.3,9.7 49.2,9.8 | 49.2,9.8 47.7,9.8 47.7,9.9 47.8,10 48.9,10 49,9.9 49,10 | 49,10 48.9,10.1 | 47.8,10.1 48.9,10.1 | 49,10 49.2,9.8 | 58,10.5 58,10.4 | 58,10.4 58,10.3 57.4,9.7 | 57.4,9.7 57.4,9.8 | 57.4,9.8 58,10.4 | 58.5,9.7 58.9,9.7 | 58.9,9.7 59.2,9.7 | 59.2,9.7 59.2,10.3 58.1,10.3 57.6,9.8 58.9,9.8 59.1,10 | 59.1,10 59,10 | 59,9.8 59,10 | 59,10 59.1,10.1 58,10.1 57.9,10 58.8,10 58.9,9.9 | 18.4,9.9 23.7,9.9 | 23.7,9.9 23.8,9.8 | 23.8,9.8 23.9,9.7 | 17.2,10.1 23.5,10.1 23.7,9.9 | 23.8,9.8 19,9.8 18.3,10.5 | 28.5,9.9 33.4,9.9 | 33.4,9.9 33.6,9.7 | 28.4,10.1 33.2,10.1 33.4,9.9 | 38.7,10 43.6,10 | 43.6,10 43.9,9.7 | 43.9,9.7 43.7,9.7 | 43.7,9.7 43.6,9.8 39.1,9.8 | 39.1,9.8 39,9.8 | 38.7,10 38.5,10.2 43.4,10.2 43.6,10 | 48.9,10.1 53.7,10.1 | 53.7,10.1 54.1,9.7 53.9,9.7 | 53.9,9.7 53.7,9.9 49.3,9.9
  Top 0.2: 48.7,10.6 49,10.3 | 49,10.3 53.5,10.3 53.7,10.1 | 60.6,9.8 59,9.8 | 59,9.8 58.9,9.7 | 59.2,9.7 60.9,9.7 60.9,11.4 60.7,11.6 59.4,11.6 59.3,11.5 | 59.2,11.1 59.2,11 | 59.2,11 59.2,10.4 | 59.2,10.4 59.2,10.1 | 59.2,10.1 59.4,9.9 60.5,9.9 60.7,10.1 | 60.7,10.1 60.7,10.3 | 60.7,10.4 60.7,10.5 | 60.7,10.5 60.7,10.8 | 60.7,11 60.7,11.5 | 60.7,10.1 60.7,9.9 60.6,9.8 | 60.6,9.8 60.6,10.1 59.2,10.1 | 59.2,10.1 59.1,10 | 59.1,10 59.1,10.3 | 59.1,10.3 59.2,10.4 | 59.2,10.4 60.7,10.4 | 60.7,10.4 60.7,10.3 | 60.7,10.3 59.1,10.3 | 59.1,10.3 59,10.2 59,10.6 59.1,10.7 60.8,10.7 60.8,10.6 60.7,10.5 | 60.7,10.5 59,10.5 58.9,10.6 58.9,10.7 59.2,11 | 59.2,11 60.7,11 | 60.7,11 60.7,10.8 | 60.7,10.8 58.9,10.8 58.9,10.9 59.3,11.3 60.6,11.3 60.6,11.1 59.2,11.1 | 59.2,11.1 59.2,11.4 59.3,11.5 | 59.3,11.5 60.5,11.5 60.6,11.4
N$120
  Top 0.2: 54.1,13 54.3,12.8 | 54.6,12.6 54.3,12.8 | 54.3,12.8 54.3,12.9 54.4,13 54.4,12.9 54.5,12.8
N$121  (2 unrouted)
  Top 0.2: 58.5,14.3 57.7,14.3 57.6,14.2 57.6,12.9 | 48.9,13.1 53.9,13.1 | 53.9,13.1 54.5,13.1 | 53.9,13.1 53.9,13 54.6,12.3 | 48.3,14.1 48.3,14.2 48.4,14.3 49.1,14.3 49.3,14.1 53.8,14.1 54.6,13.3 | 38.7,13.5 38.7,13.2 | 38.7,13.2 38.7,12.9 43.7,12.9 44.2,12.4 44.3,12.4 | 44.3,12.4 44.4,12.4 | 44.4,12.4 44.2,12.6 44.1,12.6 43.7,13 38.8,13 38.6,13.2 | 38.6,13.2 38.7,13.2 | 38.7,13.2 43.8,13.2 43.8,13.3 39,13.3 38.8,13.5 | 38.6,13.2 38.8,13.4 44,13.4 44.4,13 | 28.5,14.2 28.6,14.3 28.8,14.3 29,14.1 33.3,14.1 33.84,13.56 | 5.1,14.8 4.9,14.8 4.5,15.2 | 4.4,15.3 6,15.3 6.1,15.2 6.1,14.8 6.4,14.5 12.6,14.5 13.5,13.6 | 4.6,15.2 4.5,15.2 | 4.5,15.2 4.4,15.3 | 4.4,15.3 4.4,13.4 5.9,13.4 6.4,12.9 13.4,12.9 14,12.3 16,12.3 16.1,12.4 | LED1.7 58.33,13.4 57.9,13.4 57.4,12.9 57.6,12.9 | R5C.1 5.2,13.56 LED6.7 13.55,13.56 13.8,13.31 13.8,12.65 14.05,12.4 16.1,12.4 | 54.65,12.3 54.6,12.65 54.6,13.3 | 54.6,13.3 54.6,13.31 54.35,13.56 LED2.7 47.73,13 47.4,13.1 | 44.65,12.4 44.4,12.65 44.4,13 | 44.4,13 44.4,13.3 | 44.4,13.3 44.4,13.31 44.15,13.56 LED3.7 37.63,13.1 37.3,13.1 | 33.84,13.56 34.2,13.2 34.2,12.65 34.45,12.4 36.5,12.4 | 33.84,13.56 LED4.7 27.4,13.56 26.34,12.4 26.3,12.4 | 24,13.3 24,12.65 24.25,12.4 24.3,12.4 | 24,13.3 24,13.31 23.75,13.56 LED5.7 17.53,13.4 17.1,13.4 | 16.1,12.4 16.6,12.9 | 17.1,13.4 17.3,13.6 | 17.6,12.9 16.7,12.9 | 16.6,12.9 16.7,12.9 | 16.7,12.9 16.9,13.1 | 17.9,14.3 23,14.3 24,13.3 | 24.3,12.4 25.9,12.4 | 25.9,12.4 26.3,12.4 | 27.2,13.3 27.3,13.4 | 23.9,12.9 23.9,12.8 24.3,12.4 | 18.3,12.9 23.4,12.9 24,12.3 26,12.3 | 26,12.3 26.2,12.3 | 26.2,12.3 26.3,12.4 | 26.3,12.4 26.8,12.9 | 26.8,12.9 27,13.1 | 27,13.1 27.2,13.3
  Top 0.2: 27.2,13.3 27.2,13.1 27.4,12.9 27,12.9 | 26.8,12.9 27,12.9 | 27,12.9 27.1,13 | 25.9,12.4 26,12.3 | 26.2,12.3 26.3,12.3 27.3,13.3 | 16.6,12.9 17.1,13.4 | 27,13.1 27,14.3 27.5,14.3 | 36.5,12.4 37,12.9 | 37,12.9 37.1,13 | 37.1,13 37.2,13.1 | 37.2,13.1 37.3,13.1 | 38.1,13.5 37.6,13.5 37.2,13.1 | 37.1,13 37.2,13 | 37.2,13 37.7,13 37.8,12.9 37,12.9 | 36.5,12.4 36.6,12.4 37.2,13 | 37.3,13.1 37.3,14.3 38.9,14.3 39.3,13.9 43.8,13.9 44.4,13.3 | 44.4,13.3 44.2,13.3 43.8,13.7 38.9,13.7 38.9,14 | 38.9,14.1 38.9,14 | 38.9,14 39.1,13.8 39.3,13.8 | 44.65,12.4 46.7,12.4 47.2,12.9 | 47.2,12.9 47.4,13.1 | 44.4,13 44.2,13 | 44.2,13 44.1,13 43.9,13.2 43.8,13.1 44.3,12.6 44.3,12.9 44.2,13 | 44.2,13 43.9,13.3 43.9,12.8 44.3,12.4 | 44.4,12.4 44.65,12.4 | 47.8,13.1 47.4,13.1 | 47.4,13.1 47.6,13.3 47.9,13 47.8,13 47.7,12.9 47.2,12.9 | 57.6,12.9 60.1,12.9 60.1,14.3 59.2,14.3 59.2,13.2 59.3,13.1 60,13.1 60,14 | 60,14 60,14.1 59.3,14.1 59.3,13.3 59.4,13.2 59.5,13.2 | 59.5,13.2 59.9,13.2 59.9,13.9 60,14 | 60,14 59.8,14 | 59.6,14 59.5,14 59.4,13.9 59.4,13.8 | 59.4,13.8 59.4,13.3 59.5,13.2 | 59.5,13.2 59.5,13.4 59.6,13.5 | 59.6,13.5 59.8,13.7 59.8,13.4 59.7,13.3 59.7,13.9 59.8,14 | 59.8,14 59.6,14 | 59.6,14 59.4,13.8 | 59.4,13.8 59.6,13.8 59.6,13.5
N$122
  Top 0.2: 61.7,12.1 62.2,11.6
N$123
  Top 0.2: 63.3,9.8 61.9,9.8 | 61.9,9.8 61.8,9.7 | 61.8,9.7 62.9,9.7 63,9.6 | 61.8,9.7 61.8,10.6 62.1,10.6 | 64,10.2 64,8.5 62.8,7.3 | 62.8,7.3 62.8,9.4 | 62.8,9.4 62.5,9.7 | 62.5,9.7 62.3,9.9 62.3,10.5 64.6,10.5 | 64.6,10.5 64.6,7.1 63,7.1 62.8,7.3 | 62.8,9.4 62.8,9.6 | 62.8,9.6 62.8,9.7 62.5,10 | 62.5,10 62.5,10.2 62.4,10.3 | 62.4,10.3 63.8,10.3 63.9,10.2 63.4,10.2 63.1,9.9 62.8,9.9 62.6,10.1 | 62.6,10.1 62.7,10.1 62.7,10 63.9,8.8 | 64.2,10 64.2,10.1 64.6,10.5 | 64.6,10.5 64.6,10.6 62.3,10.6 | 62.3,10.6 62.3,10.4 62.4,10.3 | 62.6,10.4 62.6,10.1 | 62.6,10.1 62.5,10 | 62.5,10 62.5,9.7 | 62.5,9.7 62.7,9.7 62.8,9.6 | 62.3,10.6 62.1,10.6 | 62.1,10.6 61.9,10.4 61.9,10.3 | 61.9,9.8 61.9,10.3 | 61.9,10.3 62,10.4 62.1,10.4 62.2,10.5 62.2,10 62.1,9.9 62.1,10.3
N$124
  Top 0.2: 65.5,13.1 61.1,13.1 61.1,13.3 | 61.1,13.3 61.1,13.5 | 61.1,13.5 61.1,13.7 | 61.1,13.9 61.1,14.3 64.1,14.3 64.2,14.2 64.2,13.9 64.7,13.4 | 64.7,13.4 64.9,13.2 61.2,13.2 61.1,13.3 | 61.1,13.3 64.6,13.3 64.7,13.4 | 64.7,13.4 61.2,13.4 61.1,13.5 | 26,14.7 25.7,14.7 | 14.8,14.1 14.6,14.1 14.4,14.3 14.4,14.8 15.7,14.8 15.8,14.7 15.8,14.3 15.7,14.2 15.7,14.4 16.1,14.8 | LED1.4 66.1,14.8 | 61.1,14.8 60.7,14.8 | 60.7,14.8 57.3,14.8 | 57.1,14.8 55.91,14.8 LED2.4 55.9,14.8 49.5,14.8 | 49.5,14.8 47,14.8 | 47,14.8 45.71,14.8 | 45.71,14.8 LED3.4 45.7,14.8 39.3,14.8 | 39.3,14.8 36.7,14.8 | 36.7,14.8 35.51,14.8 | 35.51,14.8 LED4.4 35.5,14.8 29.2,14.8 | 29.2,14.8 26.5,14.8 | 26.5,14.8 26.4,14.8 | 26.2,14.8 25.31,14.8 LED5.4 25.3,14.8 24,14.8 | 24,14.8 23.7,14.8 | 23.6,14.8 16.1,14.8 | 15.9,14.8 15.11,14.8 LED6.4 | 66.1,14.8 67.6,14.8 | 67.6,14.8 68.3,14.8 R3E.1 | 16.1,14.8 15.9,14.8 | 15.9,14.8 15.5,14.4 14.7,14.4 14.6,14.5 | 14.6,14.5 14.6,14.6 | 14.6,14.6 14.7,14.6 | 15.6,14.6 14.7,14.6 | 14.7,14.6 14.6,14.7 14.6,14.6 | 14.6,14.5 14.5,14.4 | 25,13.9 24.9,13.9 24,14.8 | 25.6,13.9 25.6,14 26.4,14.8 | 26.4,14.8 26.2,14.8 | 26.2,14.8 25.9,14.5 | 25.7,14.2 25.9,14.2 26.5,14.8 | 24.3,14.7 25.7,14.7 | 25.7,14.7 25.9,14.5 | 25.9,14.5 24.4,14.5 | 24.8,13.5 24.8,13.6 23.6,14.8 | 23.6,14.8 23.7,14.8 | 23.7,14.8 24.5,14 | 29.2,14.8 29.3,14.7 34.1,14.7 34.9,13.9 35.8,13.9 36.7,14.8 | 35.51,14.8 34.6,14.8 34.4,14.6 34.3,14.7 36.4,14.7 36.4,14.6 36.2,14.4 34.5,14.4 34.4,14.5 36.1,14.5 36.2,14.6 35.4,14.6 35,14.2 | 39.3,14.8 39.4,14.7 44.2,14.7 45.1,13.8 46,13.8 47,14.8 | 45.71,14.8 44.6,14.8 44.4,14.6 44.6,14.6 | 46.7,14.6 44.6,14.6 | 44.6,14.6 44.5,14.5 44.9,14.5
  Top 0.2: 46.5,14.5 44.9,14.5 | 44.9,14.5 44.7,14.3 44.8,14.3 45,14.1 | 49.5,14.8 49.6,14.7 54.4,14.7 55.2,13.9 56.2,13.9 | 56.6,13.9 56.2,13.9 | 56.2,13.9 56.1,14 | 56.2,13.9 56.4,13.7 56.4,13.9 56.5,14 | 57.3,14.8 57.1,14.8 | 57.1,14.8 56.6,14.3 | 56.6,14.3 56.6,14.4 | 56.6,14.4 56.8,14.6 54.6,14.6 55,14.2 55,14.3 54.8,14.5 56.5,14.5 56.6,14.4 | 56.6,14.3 56.6,13.8 56.5,13.7 56.5,14 | 56.5,14 57.3,14.8 | 60.7,14.8 60.9,14.6 | 61,14.5 63.7,14.5 65.3,12.9 67,12.9 67.6,13.5 69.2,13.5 69.2,15.4 67.7,15.4 67.6,15.3 67.6,14.8 | 66.1,14.8 61.1,14.8 | 61.1,14.8 61,14.7 67.6,14.7 | 67.7,14.7 67.6,14.7 | 67.6,14.7 67.4,14.5 63.8,14.5 63.7,14.6 67.5,14.6 67.7,14.4 64.1,14.4 64,14.3 67.7,14.3 67.8,14.4 67.8,14.2 66.9,14.2 | 66.9,14.2 64.4,14.2 64.3,14.1 | 64.2,14.1 64.3,14.1 | 64.3,14.1 64.4,14 67.8,14 67.8,13.8 64.9,13.8 | 64.9,13.8 64.5,13.8 64.7,13.6 64.9,13.6 | 64.9,13.6 67.4,13.6 | 67.6,13.6 67.4,13.6 | 67.4,13.6 67.3,13.5 | 67.2,13.4 66.9,13.1 66.9,13.3 67,13.4 67.2,13.4 | 67.2,13.4 67.3,13.5 | 67.3,13.5 64.9,13.5 65.3,13.1 65.3,13.3 65.2,13.4 66.5,13.4 66.9,13 66,13 65.8,13.2 | 60.9,14.7 60.9,14.6 | 60.9,14.6 61,14.5 | 61,14.5 61,12.9 66.9,12.9 67.5,13.5 | 61.1,13.5 64.8,13.5 64.9,13.6 | 64.9,13.6 64.8,13.7 61.1,13.7 | 61.1,13.7 61.1,13.9 | 61.1,13.9 64.8,13.9 64.9,13.8 | 64.9,13.8 64.9,14.1 61.2,14.1 | 66.9,14.2 66.9,14.3 67.8,15.2
N$125
  Top 0.2: 65.6,23.3 65.6,23.2 | 65.6,23.2 65,23.2 65,26.4 65.3,26.7 | 72.6,15.7 72.6,26.45 72.35,26.7 66.4,26.7 | 72.6,15.7 72.6,14.65 72.35,14.4 R3E.2 | 66.4,26.7 65.99,26.7 | 65.99,26.7 65.74,26.45 JP16.3 | 65.3,26.7 65.6,26.7 | 65.6,26.7 65.99,26.7 | 66.4,26.7 66.4,26.6 | 66.4,26.6 66.4,26.5 | 66.4,26.5 66.4,23.2 | 66.4,23.2 65.6,23.2 | 66.4,23.2 66.5,23.2 66.5,26.4 66.7,26.6 66.4,26.6 | 65.3,26.7 65.5,26.9 72.8,26.9 72.9,26.8 72.9,13.5 72.8,13.4 70.5,13.4 70.5,15.4 72.3,15.4 72.6,15.7 | 72.6,15.7 72.8,15.5 72.8,13.6 72.7,13.5 71.9,13.5 71.8,13.6 71.8,15 72.1,15.3 72.4,15.3 72.8,15.7 72.7,15.7 72,15 72,13.7 72.1,13.6 72.2,13.6 | 72.3,13.6 72.6,13.6 72.7,13.7 | 72.7,13.7 72.7,15 72.5,15.2 72.4,15.2 72.1,14.9 72.1,13.7 72.2,13.6 | 72.2,13.6 72.3,13.6 | 72.3,13.6 72.6,13.9 72.6,14.9 72.4,15.1 72.4,13.8 72.3,13.7 72.3,14.8 72.2,14.9 72.2,14.2 72.7,13.7 | 66.4,26.5 66,26.5 | 65.8,26.5 65.4,26.5 | 65.4,26.5 65.3,26.5 65.1,26.3 | 65.4,26.5 65.4,23.3 65.2,23.3 65.2,26.3 65.4,26.5 | 65.4,26.5 65.6,26.7 | 65.6,26.7 65.6,23.3 | 65.6,23.3 65.8,23.3 65.8,26.5 | 65.8,26.5 66,26.5 | 66,26.5 66,23.4 65.9,23.3 66.2,23.3 66.2,26.6
N$126
  Top 0.2: 13.8,18.9 13.8,19.6 14,19.8 16,19.8 17.2,18.6
N$127
  Top 0.2: 1.5,18.6 1.5,16.9 | 1.5,16.9 1.3,16.9 | 1.5,16.9 1.6,16.9 1.6,18.7 1.5,18.7
N$128
  Top 0.2: 1.7,15.1 0.7,15.1 0.5,15.3 1.4,15.3 1.5,15.2 1.6,15.3 1.6,13.6 0.5,13.6 | 0.5,13.7 0.5,15.2 | 0.5,13.6 0.5,13.5 | 0.5,13.6 0.5,13.7 | 0.5,13.7 0.6,13.8 1.5,13.8 1.5,15 1.2,15 | 60.8,26.1 59.8,26.1 | 59.8,26.1 59.8,25.8 | 59.8,25.8 59.8,23.2 60.7,23.2 | 60.9,23.2 61.4,23.2 | 61.4,23.2 61.4,27.7 | 61.4,27.7 0.3,27.7 0.3,13.4 3.2,13.4 3.2,15.4 0.5,15.4 | 60.1,25.5 59.8,25.8 | 59.8,26.1 59.8,27.3 59.5,27.6 61.1,27.6 61.3,27.4 61.3,23.4 61.2,23.3 61.2,27.3 61.1,27.4 60.7,27.4 | 60.5,27.4 60.2,27.4 | 60.2,27.4 59.9,27.4 59.9,23.3 60.1,23.3 | 60.1,23.3 60.2,23.3 | 60.2,23.3 60.2,27.4 | 60.2,27.4 60.1,27.3 60.1,23.3 | 60.2,23.3 60.3,23.3 | 60.3,23.3 60.5,23.3 60.5,23.4 | 60.5,24.9 60.5,25.5 | 60.5,26.2 60.5,27.1 60.4,27.2 60.4,23.4 60.3,23.3 | 60.3,23.3 60.3,25.7 | 60.3,26.6 60.3,27.2 60.5,27.4 | 60.5,27.4 60.7,27.4 | 60.7,27.4 60.8,27.3 60.8,23.3 60.7,23.2 | 60.7,23.2 60.9,23.2 | 60.9,23.2 60.9,27.1 61.1,27.3 61,27.3 61,23.4 61.1,23.3 60.6,23.3 60.5,23.4 | R5C.2 0.95,14.4 0.7,14.65 | 60.6,25 60.6,27.4 60.7,27.5 | 60.6,25 60.6,24.76 | 60.6,24.76 JP16.5 | 0.7,14.8 0.7,14.9 | 0.7,14.9 0.7,15.2 0.5,15.4 | 0.5,15.4 0.5,15.6 | 0.5,15.8 0.5,27.5 | 0.5,27.6 0.5,27.5 | 0.5,27.5 59.2,27.5 | 59.2,27.5 59.4,27.5 | 59.4,27.5 60.7,27.5 | 60.7,27.5 61.3,27.5 | 60.5,23.4 60.5,24.9 | 60.5,24.9 60.6,25 | 60.6,24.76 60.6,23.4 | 61.4,27.7 61.5,27.7 61.5,23.2 61.4,23.2 | 59.4,27.5 60.3,26.6 | 60.3,26.6 60.3,25.7 | 60.3,25.7 60.5,25.5 | 60.5,25.5 60.5,26.2 | 60.5,26.2 59.2,27.5 | 1.2,15 0.8,15 0.7,14.9 | 0.7,14.65 0.7,14 | 0.7,14 0.8,13.9 | 0.8,13.9 0.7,13.9 | 0.8,13.9 1.3,13.9 1.4,14 1.4,14.8 1.3,14.9 1.1,14.9 | 1.1,14.9 0.9,14.9 | 0.9,14.9 0.8,14.9 0.7,14.8 | 0.7,14.8 0.7,14.65
  Top 0.2: 0.7,14 0.6,13.9 0.6,14.1 1.3,14.8 1.3,14.1 1.2,14 | 1.2,14 0.8,14 0.8,14.8 0.9,14.9 | 0.9,14.9 0.9,14.4 1.1,14.2 1,14.1 1,14.8 1.1,14.9 | 1.1,14.9 1.1,14.1 1.2,14 | 1.2,15 1.2,15.1 0.5,15.8 | 0.5,15.8 0.5,15.6 | 0.5,15.6 0.6,15.5
N$129
  Top 0.2: 0.4,27 0.4,27.1 0.9,27.6
N$130
  Top 0.2: 13.8,19.7 12.8,19.7 12.4,19.3 13.7,19.3 13.7,19.5 12.7,19.5
N$131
